DATA_BLOCK "IMAC_MOTOR2_RECORD"
TITLE =  MOTOR2_RECORD
AUTHOR : HottendU
FAMILY : IMAC
VERSION : 0.2


  STRUCT
   MOTOR2_No001 : STRUCT
    System : WORD ;
    CmdOS : WORD ;
    MirrorCmdOS : WORD ;
    Test : WORD ;
    AlarmOS : WORD ;
    StatusOS : WORD ;
    SysStatusOS : WORD ;
    Status1 : WORD ;
    Status2 : WORD ;
    Status3 : BYTE ;
    InputEdges : BYTE ;
    AutoEdges : WORD ;
    DataTimeCmd : STRUCT
     StartTime : DINT ;
     StartEdge : BOOL ;
    END_STRUCT ;
    DataTimeChg12 : STRUCT
     StartTime : DINT ;
     StartEdge : BOOL ;
    END_STRUCT ;
    DataTimeChg21 : STRUCT
     StartTime : DINT ;
     StartEdge : BOOL ;
    END_STRUCT ;
    DataTimeBlackout : STRUCT
     StartTime : DINT ;
     StartEdge : BOOL ;
    END_STRUCT ;
    DataTimeActFault : STRUCT
     StartTime : DINT ;
     StartEdge : BOOL ;
    END_STRUCT ;
    DataTimeExtFault : STRUCT
     StartTime : DINT ;
     StartEdge : BOOL ;
    END_STRUCT ;
    DataTimeFeedback : STRUCT
     StartTime : DINT ;
     StartEdge : BOOL ;
    END_STRUCT ;
    DataTimeAutoAl : STRUCT
     StartTime : DINT ;
     StartEdge : BOOL ;
    END_STRUCT ;
    PCONF : STRUCT 	//// PCONF MOTOR2 - Instance 001
     Modeswitches : STRUCT
      M0_ConstantOut : BOOL  := TRUE;	// Constant Output MST1 MST2 MSTO (1); Feedback depended Output Anst. (0)
      M1_AutoManLoc : BOOL  := TRUE;	// AUTO/ MANUAL/ LOCAL (1); MANUAL/ LOCAL (0)
      M2_NoActFeedFault : BOOL ;	// No Action- and Non-Feedback fault(1),
      M3_NoStopIfFault : BOOL  := TRUE;	// No Stop-Signal if Failure occurs (1)
      M4_RestrtAftBlack : BOOL  := TRUE;	// Restart after Blackout (1)
      M5_ResetOSonly : BOOL  := TRUE;	// Reset Alarm only with RESET from OS (1); RESET and START/STOP-Command (0)
      M6_CmdTimeDly : BOOL ;	// Command Time Delay aktiv (1)
      M7_Chg12viaStop : BOOL ;	// Change from 1->2 via STOP(1)
      M8_Chg21viaStop : BOOL ;	// Change from 2->1 via STOP(1)
      M9_StopIfAutoFail : BOOL ;	// NO AVAIL Direct Stop if Auto Failure (1)
      M10_LockBlockCmd : BOOL ;	// Lock blocksCommands
      sw11 : BOOL ;
      sw12 : BOOL ;
      sw13 : BOOL ;
      sw14 : BOOL ;
      sw15 : BOOL ;	//
     END_STRUCT ;
     DlyTCmd : TIME ;	// Setpoint Command time delay
     DlyTBlackout : TIME  := T#30S;	// Setpoint blackout time delay
     DlyTExtFault : TIME  := T#2S;	// Setpoint external fault delay
     DlyTFeedback : TIME  := T#1S;	// Setpoint feedback fault delay
     DlyTActFault : TIME  := T#5S;	// Setpoint Action Fault delay
     DlyTAutoAl : TIME  := T#3S;	// Setpoint auto alarm delay
     DlyTRestart : TIME ;	// No AVAIL Setpoint restart after blackout delay
     DlyTChg12 : TIME  := T#500MS;	// Setpoint Waiting Delay 1->2
     DlyTChg21 : TIME  := T#500MS;	// Setpoint Waiting Delay 2->1
    END_STRUCT ;
   END_STRUCT ;
   MOTOR2_No002 : STRUCT
    System : WORD ;
    CmdOS : WORD ;
    MirrorCmdOS : WORD ;
    Test : WORD ;
    AlarmOS : WORD ;
    StatusOS : WORD ;
    SysStatusOS : WORD ;
    Status1 : WORD ;
    Status2 : WORD ;
    Status3 : BYTE ;
    InputEdges : BYTE ;
    AutoEdges : WORD ;
    DataTimeCmd : STRUCT
     StartTime : DINT ;
     StartEdge : BOOL ;
    END_STRUCT ;
    DataTimeChg12 : STRUCT
     StartTime : DINT ;
     StartEdge : BOOL ;
    END_STRUCT ;
    DataTimeChg21 : STRUCT
     StartTime : DINT ;
     StartEdge : BOOL ;
    END_STRUCT ;
    DataTimeBlackout : STRUCT
     StartTime : DINT ;
     StartEdge : BOOL ;
    END_STRUCT ;
    DataTimeActFault : STRUCT
     StartTime : DINT ;
     StartEdge : BOOL ;
    END_STRUCT ;
    DataTimeExtFault : STRUCT
     StartTime : DINT ;
     StartEdge : BOOL ;
    END_STRUCT ;
    DataTimeFeedback : STRUCT
     StartTime : DINT ;
     StartEdge : BOOL ;
    END_STRUCT ;
    DataTimeAutoAl : STRUCT
     StartTime : DINT ;
     StartEdge : BOOL ;
    END_STRUCT ;
    PCONF : STRUCT 	//// PCONF MOTOR1 - Instance 002
     Modeswitches : STRUCT
      M0_ConstantOut : BOOL  := TRUE;	// Constant Output MST1 MST2 MSTO (1); Feedback depended Output Anst. (0)
      M1_AutoManLoc : BOOL  := TRUE;	// AUTO/ MANUAL/ LOCAL (1); MANUAL/ LOCAL (0)
      M2_NoActFeedFault : BOOL ;	// No Action- and Non-Feedback fault(1),
      M3_NoStopIfFault : BOOL  := TRUE;	// No Stop-Signal if Failure occurs (1)
      M4_RestrtAftBlack : BOOL  := TRUE;	// Restart after Blackout (1)
      M5_ResetOSonly : BOOL  := TRUE;	// Reset Alarm only with RESET from OS (1); RESET and START/STOP-Command (0)
      M6_CmdTimeDly : BOOL ;	// Command Time Delay aktiv (1)
      M7_Chg12viaStop : BOOL ;	// Change from 1->2 via STOP(1)
      M8_Chg21viaStop : BOOL ;	// Change from 2->1 via STOP(1)
      M9_StopIfAutoFail : BOOL ;	// NO AVAIL Direct Stop if Auto Failure (1)
      M10_LockBlockCmd : BOOL ;	// Lock blocksCommands
      sw11 : BOOL ;
      sw12 : BOOL ;
      sw13 : BOOL ;
      sw14 : BOOL ;
      sw15 : BOOL ;	//
     END_STRUCT ;
     DlyTCmd : TIME ;	// Setpoint Command time delay
     DlyTBlackout : TIME  := T#30S;	// Setpoint blackout time delay
     DlyTExtFault : TIME  := T#2S;	// Setpoint external fault delay
     DlyTFeedback : TIME  := T#1S;	// Setpoint feedback fault delay
     DlyTActFault : TIME  := T#5S;	// Setpoint Action Fault delay
     DlyTAutoAl : TIME  := T#3S;	// Setpoint auto alarm delay
     DlyTRestart : TIME ;	// No AVAIL Setpoint restart after blackout delay
     DlyTChg12 : TIME  := T#500MS;	// Setpoint Waiting Delay 1->2
     DlyTChg21 : TIME  := T#500MS;	// Setpoint Waiting Delay 2->1
    END_STRUCT ;
   END_STRUCT ;
   MOTOR2_No003 : STRUCT
    System : WORD ;
    CmdOS : WORD ;
    MirrorCmdOS : WORD ;
    Test : WORD ;
    AlarmOS : WORD ;
    StatusOS : WORD ;
    SysStatusOS : WORD ;
    Status1 : WORD ;
    Status2 : WORD ;
    Status3 : BYTE ;
    InputEdges : BYTE ;
    AutoEdges : WORD ;
    DataTimeCmd : STRUCT
     StartTime : DINT ;
     StartEdge : BOOL ;
    END_STRUCT ;
    DataTimeChg12 : STRUCT
     StartTime : DINT ;
     StartEdge : BOOL ;
    END_STRUCT ;
    DataTimeChg21 : STRUCT
     StartTime : DINT ;
     StartEdge : BOOL ;
    END_STRUCT ;
    DataTimeBlackout : STRUCT
     StartTime : DINT ;
     StartEdge : BOOL ;
    END_STRUCT ;
    DataTimeActFault : STRUCT
     StartTime : DINT ;
     StartEdge : BOOL ;
    END_STRUCT ;
    DataTimeExtFault : STRUCT
     StartTime : DINT ;
     StartEdge : BOOL ;
    END_STRUCT ;
    DataTimeFeedback : STRUCT
     StartTime : DINT ;
     StartEdge : BOOL ;
    END_STRUCT ;
    DataTimeAutoAl : STRUCT
     StartTime : DINT ;
     StartEdge : BOOL ;
    END_STRUCT ;
    PCONF : STRUCT 	//// PCONF MOTOR1 - Instance 003
     Modeswitches : STRUCT
      M0_ConstantOut : BOOL  := TRUE;	// Constant Output MST1 MST2 MSTO (1); Feedback depended Output Anst. (0)
      M1_AutoManLoc : BOOL  := TRUE;	// AUTO/ MANUAL/ LOCAL (1); MANUAL/ LOCAL (0)
      M2_NoActFeedFault : BOOL ;	// No Action- and Non-Feedback fault(1),
      M3_NoStopIfFault : BOOL  := TRUE;	// No Stop-Signal if Failure occurs (1)
      M4_RestrtAftBlack : BOOL  := TRUE;	// Restart after Blackout (1)
      M5_ResetOSonly : BOOL  := TRUE;	// Reset Alarm only with RESET from OS (1); RESET and START/STOP-Command (0)
      M6_CmdTimeDly : BOOL ;	// Command Time Delay aktiv (1)
      M7_Chg12viaStop : BOOL ;	// Change from 1->2 via STOP(1)
      M8_Chg21viaStop : BOOL ;	// Change from 2->1 via STOP(1)
      M9_StopIfAutoFail : BOOL ;	// NO AVAIL Direct Stop if Auto Failure (1)
      M10_LockBlockCmd : BOOL ;	// Lock blocksCommands
      sw11 : BOOL ;
      sw12 : BOOL ;
      sw13 : BOOL ;
      sw14 : BOOL ;
      sw15 : BOOL ;	//
     END_STRUCT ;
     DlyTCmd : TIME ;	// Setpoint Command time delay
     DlyTBlackout : TIME  := T#30S;	// Setpoint blackout time delay
     DlyTExtFault : TIME  := T#2S;	// Setpoint external fault delay
     DlyTFeedback : TIME  := T#1S;	// Setpoint feedback fault delay
     DlyTActFault : TIME  := T#5S;	// Setpoint Action Fault delay
     DlyTAutoAl : TIME  := T#3S;	// Setpoint auto alarm delay
     DlyTRestart : TIME ;	// No AVAIL Setpoint restart after blackout delay
     DlyTChg12 : TIME  := T#500MS;	// Setpoint Waiting Delay 1->2
     DlyTChg21 : TIME  := T#500MS;	// Setpoint Waiting Delay 2->1
    END_STRUCT ;
   END_STRUCT ;
   MOTOR2_No0004 : STRUCT
    System : WORD ;
    CmdOS : WORD ;
    MirrorCmdOS : WORD ;
    Test : WORD ;
    AlarmOS : WORD ;
    StatusOS : WORD ;
    SysStatusOS : WORD ;
    Status1 : WORD ;
    Status2 : WORD ;
    Status3 : BYTE ;
    InputEdges : BYTE ;
    AutoEdges : WORD ;
    DataTimeCmd : STRUCT
     StartTime : DINT ;
     StartEdge : BOOL ;
    END_STRUCT ;
    DataTimeChg12 : STRUCT
     StartTime : DINT ;
     StartEdge : BOOL ;
    END_STRUCT ;
    DataTimeChg21 : STRUCT
     StartTime : DINT ;
     StartEdge : BOOL ;
    END_STRUCT ;
    DataTimeBlackout : STRUCT
     StartTime : DINT ;
     StartEdge : BOOL ;
    END_STRUCT ;
    DataTimeActFault : STRUCT
     StartTime : DINT ;
     StartEdge : BOOL ;
    END_STRUCT ;
    DataTimeExtFault : STRUCT
     StartTime : DINT ;
     StartEdge : BOOL ;
    END_STRUCT ;
    DataTimeFeedback : STRUCT
     StartTime : DINT ;
     StartEdge : BOOL ;
    END_STRUCT ;
    DataTimeAutoAl : STRUCT
     StartTime : DINT ;
     StartEdge : BOOL ;
    END_STRUCT ;
    PCONF : STRUCT 	//// PCONF MOTOR1 - Instance 004
     Modeswitches : STRUCT
      M0_ConstantOut : BOOL ;	// Constant Output MST1 MST2 MSTO (1); Feedback depended Output Anst. (0)
      M1_AutoManLoc : BOOL ;	// AUTO/ MANUAL/ LOCAL (1); MANUAL/ LOCAL (0)
      M2_NoActFeedFault : BOOL ;	// No Action- and Non-Feedback fault(1),
      M3_NoStopIfFault : BOOL ;	// No Stop-Signal if Failure occurs (1)
      M4_RestrtAftBlack : BOOL ;	// Restart after Blackout (1)
      M5_ResetOSonly : BOOL ;	// Reset Alarm only with RESET from OS (1); RESET and START/STOP-Command (0)
      M6_CmdTimeDly : BOOL ;	// Command Time Delay aktiv (1)
      M7_Chg12viaStop : BOOL ;	// Change from 1->2 via STOP(1)
      M8_Chg21viaStop : BOOL ;	// Change from 2->1 via STOP(1)
      M9_StopIfAutoFail : BOOL ;	// NO AVAIL Direct Stop if Auto Failure (1)
      M10_LockBlockCmd : BOOL ;	// Lock blocksCommands
      sw11 : BOOL ;
      sw12 : BOOL ;
      sw13 : BOOL ;
      sw14 : BOOL ;
      sw15 : BOOL ;	//
     END_STRUCT ;
     DlyTCmd : TIME ;	// Setpoint Command time delay
     DlyTBlackout : TIME ;	// Setpoint blackout time delay
     DlyTExtFault : TIME ;	// Setpoint external fault delay
     DlyTFeedback : TIME ;	// Setpoint feedback fault delay
     DlyTActFault : TIME ;	// Setpoint Action Fault delay
     DlyTAutoAl : TIME ;	// Setpoint auto alarm delay
     DlyTRestart : TIME ;	// No AVAIL Setpoint restart after blackout delay
     DlyTChg12 : TIME ;	// Setpoint Waiting Delay 1->2
     DlyTChg21 : TIME ;	// Setpoint Waiting Delay 2->1
    END_STRUCT ;
   END_STRUCT ;
   MOTOR2_No005 : STRUCT
    System : WORD ;
    CmdOS : WORD ;
    MirrorCmdOS : WORD ;
    Test : WORD ;
    AlarmOS : WORD ;
    StatusOS : WORD ;
    SysStatusOS : WORD ;
    Status1 : WORD ;
    Status2 : WORD ;
    Status3 : BYTE ;
    InputEdges : BYTE ;
    AutoEdges : WORD ;
    DataTimeCmd : STRUCT
     StartTime : DINT ;
     StartEdge : BOOL ;
    END_STRUCT ;
    DataTimeChg12 : STRUCT
     StartTime : DINT ;
     StartEdge : BOOL ;
    END_STRUCT ;
    DataTimeChg21 : STRUCT
     StartTime : DINT ;
     StartEdge : BOOL ;
    END_STRUCT ;
    DataTimeBlackout : STRUCT
     StartTime : DINT ;
     StartEdge : BOOL ;
    END_STRUCT ;
    DataTimeActFault : STRUCT
     StartTime : DINT ;
     StartEdge : BOOL ;
    END_STRUCT ;
    DataTimeExtFault : STRUCT
     StartTime : DINT ;
     StartEdge : BOOL ;
    END_STRUCT ;
    DataTimeFeedback : STRUCT
     StartTime : DINT ;
     StartEdge : BOOL ;
    END_STRUCT ;
    DataTimeAutoAl : STRUCT
     StartTime : DINT ;
     StartEdge : BOOL ;
    END_STRUCT ;
    PCONF : STRUCT 	//// PCONF MOTOR1 - Instance 005
     Modeswitches : STRUCT
      M0_ConstantOut : BOOL ;	// Constant Output MST1 MST2 MSTO (1); Feedback depended Output Anst. (0)
      M1_AutoManLoc : BOOL ;	// AUTO/ MANUAL/ LOCAL (1); MANUAL/ LOCAL (0)
      M2_NoActFeedFault : BOOL ;	// No Action- and Non-Feedback fault(1),
      M3_NoStopIfFault : BOOL ;	// No Stop-Signal if Failure occurs (1)
      M4_RestrtAftBlack : BOOL ;	// Restart after Blackout (1)
      M5_ResetOSonly : BOOL ;	// Reset Alarm only with RESET from OS (1); RESET and START/STOP-Command (0)
      M6_CmdTimeDly : BOOL ;	// Command Time Delay aktiv (1)
      M7_Chg12viaStop : BOOL ;	// Change from 1->2 via STOP(1)
      M8_Chg21viaStop : BOOL ;	// Change from 2->1 via STOP(1)
      M9_StopIfAutoFail : BOOL ;	// NO AVAIL Direct Stop if Auto Failure (1)
      M10_LockBlockCmd : BOOL ;	// Lock blocksCommands
      sw11 : BOOL ;
      sw12 : BOOL ;
      sw13 : BOOL ;
      sw14 : BOOL ;
      sw15 : BOOL ;	//
     END_STRUCT ;
     DlyTCmd : TIME ;	// Setpoint Command time delay
     DlyTBlackout : TIME ;	// Setpoint blackout time delay
     DlyTExtFault : TIME ;	// Setpoint external fault delay
     DlyTFeedback : TIME ;	// Setpoint feedback fault delay
     DlyTActFault : TIME ;	// Setpoint Action Fault delay
     DlyTAutoAl : TIME ;	// Setpoint auto alarm delay
     DlyTRestart : TIME ;	// No AVAIL Setpoint restart after blackout delay
     DlyTChg12 : TIME ;	// Setpoint Waiting Delay 1->2
     DlyTChg21 : TIME ;	// Setpoint Waiting Delay 2->1
    END_STRUCT ;
   END_STRUCT ;
   MOTOR2_No006 : STRUCT
    System : WORD ;
    CmdOS : WORD ;
    MirrorCmdOS : WORD ;
    Test : WORD ;
    AlarmOS : WORD ;
    StatusOS : WORD ;
    SysStatusOS : WORD ;
    Status1 : WORD ;
    Status2 : WORD ;
    Status3 : BYTE ;
    InputEdges : BYTE ;
    AutoEdges : WORD ;
    DataTimeCmd : STRUCT
     StartTime : DINT ;
     StartEdge : BOOL ;
    END_STRUCT ;
    DataTimeChg12 : STRUCT
     StartTime : DINT ;
     StartEdge : BOOL ;
    END_STRUCT ;
    DataTimeChg21 : STRUCT
     StartTime : DINT ;
     StartEdge : BOOL ;
    END_STRUCT ;
    DataTimeBlackout : STRUCT
     StartTime : DINT ;
     StartEdge : BOOL ;
    END_STRUCT ;
    DataTimeActFault : STRUCT
     StartTime : DINT ;
     StartEdge : BOOL ;
    END_STRUCT ;
    DataTimeExtFault : STRUCT
     StartTime : DINT ;
     StartEdge : BOOL ;
    END_STRUCT ;
    DataTimeFeedback : STRUCT
     StartTime : DINT ;
     StartEdge : BOOL ;
    END_STRUCT ;
    DataTimeAutoAl : STRUCT
     StartTime : DINT ;
     StartEdge : BOOL ;
    END_STRUCT ;
    PCONF : STRUCT 	//// PCONF MOTOR1 - Instance 006
     Modeswitches : STRUCT
      M0_ConstantOut : BOOL ;	// Constant Output MST1 MST2 MSTO (1); Feedback depended Output Anst. (0)
      M1_AutoManLoc : BOOL ;	// AUTO/ MANUAL/ LOCAL (1); MANUAL/ LOCAL (0)
      M2_NoActFeedFault : BOOL ;	// No Action- and Non-Feedback fault(1),
      M3_NoStopIfFault : BOOL ;	// No Stop-Signal if Failure occurs (1)
      M4_RestrtAftBlack : BOOL ;	// Restart after Blackout (1)
      M5_ResetOSonly : BOOL ;	// Reset Alarm only with RESET from OS (1); RESET and START/STOP-Command (0)
      M6_CmdTimeDly : BOOL ;	// Command Time Delay aktiv (1)
      M7_Chg12viaStop : BOOL ;	// Change from 1->2 via STOP(1)
      M8_Chg21viaStop : BOOL ;	// Change from 2->1 via STOP(1)
      M9_StopIfAutoFail : BOOL ;	// NO AVAIL Direct Stop if Auto Failure (1)
      M10_LockBlockCmd : BOOL ;	// Lock blocksCommands
      sw11 : BOOL ;
      sw12 : BOOL ;
      sw13 : BOOL ;
      sw14 : BOOL ;
      sw15 : BOOL ;	//
     END_STRUCT ;
     DlyTCmd : TIME ;	// Setpoint Command time delay
     DlyTBlackout : TIME ;	// Setpoint blackout time delay
     DlyTExtFault : TIME ;	// Setpoint external fault delay
     DlyTFeedback : TIME ;	// Setpoint feedback fault delay
     DlyTActFault : TIME ;	// Setpoint Action Fault delay
     DlyTAutoAl : TIME ;	// Setpoint auto alarm delay
     DlyTRestart : TIME ;	// No AVAIL Setpoint restart after blackout delay
     DlyTChg12 : TIME ;	// Setpoint Waiting Delay 1->2
     DlyTChg21 : TIME ;	// Setpoint Waiting Delay 2->1
    END_STRUCT ;
   END_STRUCT ;
   MOTOR2_No007 : STRUCT
    System : WORD ;
    CmdOS : WORD ;
    MirrorCmdOS : WORD ;
    Test : WORD ;
    AlarmOS : WORD ;
    StatusOS : WORD ;
    SysStatusOS : WORD ;
    Status1 : WORD ;
    Status2 : WORD ;
    Status3 : BYTE ;
    InputEdges : BYTE ;
    AutoEdges : WORD ;
    DataTimeCmd : STRUCT
     StartTime : DINT ;
     StartEdge : BOOL ;
    END_STRUCT ;
    DataTimeChg12 : STRUCT
     StartTime : DINT ;
     StartEdge : BOOL ;
    END_STRUCT ;
    DataTimeChg21 : STRUCT
     StartTime : DINT ;
     StartEdge : BOOL ;
    END_STRUCT ;
    DataTimeBlackout : STRUCT
     StartTime : DINT ;
     StartEdge : BOOL ;
    END_STRUCT ;
    DataTimeActFault : STRUCT
     StartTime : DINT ;
     StartEdge : BOOL ;
    END_STRUCT ;
    DataTimeExtFault : STRUCT
     StartTime : DINT ;
     StartEdge : BOOL ;
    END_STRUCT ;
    DataTimeFeedback : STRUCT
     StartTime : DINT ;
     StartEdge : BOOL ;
    END_STRUCT ;
    DataTimeAutoAl : STRUCT
     StartTime : DINT ;
     StartEdge : BOOL ;
    END_STRUCT ;
    PCONF : STRUCT 	//// PCONF MOTOR1 - Instance 007
     Modeswitches : STRUCT
      M0_ConstantOut : BOOL ;	// Constant Output MST1 MST2 MSTO (1); Feedback depended Output Anst. (0)
      M1_AutoManLoc : BOOL ;	// AUTO/ MANUAL/ LOCAL (1); MANUAL/ LOCAL (0)
      M2_NoActFeedFault : BOOL ;	// No Action- and Non-Feedback fault(1),
      M3_NoStopIfFault : BOOL ;	// No Stop-Signal if Failure occurs (1)
      M4_RestrtAftBlack : BOOL ;	// Restart after Blackout (1)
      M5_ResetOSonly : BOOL ;	// Reset Alarm only with RESET from OS (1); RESET and START/STOP-Command (0)
      M6_CmdTimeDly : BOOL ;	// Command Time Delay aktiv (1)
      M7_Chg12viaStop : BOOL ;	// Change from 1->2 via STOP(1)
      M8_Chg21viaStop : BOOL ;	// Change from 2->1 via STOP(1)
      M9_StopIfAutoFail : BOOL ;	// NO AVAIL Direct Stop if Auto Failure (1)
      M10_LockBlockCmd : BOOL ;	// Lock blocksCommands
      sw11 : BOOL ;
      sw12 : BOOL ;
      sw13 : BOOL ;
      sw14 : BOOL ;
      sw15 : BOOL ;	//
     END_STRUCT ;
     DlyTCmd : TIME ;	// Setpoint Command time delay
     DlyTBlackout : TIME ;	// Setpoint blackout time delay
     DlyTExtFault : TIME ;	// Setpoint external fault delay
     DlyTFeedback : TIME ;	// Setpoint feedback fault delay
     DlyTActFault : TIME ;	// Setpoint Action Fault delay
     DlyTAutoAl : TIME ;	// Setpoint auto alarm delay
     DlyTRestart : TIME ;	// No AVAIL Setpoint restart after blackout delay
     DlyTChg12 : TIME ;	// Setpoint Waiting Delay 1->2
     DlyTChg21 : TIME ;	// Setpoint Waiting Delay 2->1
    END_STRUCT ;
   END_STRUCT ;
   MOTOR2_No008 : STRUCT
    System : WORD ;
    CmdOS : WORD ;
    MirrorCmdOS : WORD ;
    Test : WORD ;
    AlarmOS : WORD ;
    StatusOS : WORD ;
    SysStatusOS : WORD ;
    Status1 : WORD ;
    Status2 : WORD ;
    Status3 : BYTE ;
    InputEdges : BYTE ;
    AutoEdges : WORD ;
    DataTimeCmd : STRUCT
     StartTime : DINT ;
     StartEdge : BOOL ;
    END_STRUCT ;
    DataTimeChg12 : STRUCT
     StartTime : DINT ;
     StartEdge : BOOL ;
    END_STRUCT ;
    DataTimeChg21 : STRUCT
     StartTime : DINT ;
     StartEdge : BOOL ;
    END_STRUCT ;
    DataTimeBlackout : STRUCT
     StartTime : DINT ;
     StartEdge : BOOL ;
    END_STRUCT ;
    DataTimeActFault : STRUCT
     StartTime : DINT ;
     StartEdge : BOOL ;
    END_STRUCT ;
    DataTimeExtFault : STRUCT
     StartTime : DINT ;
     StartEdge : BOOL ;
    END_STRUCT ;
    DataTimeFeedback : STRUCT
     StartTime : DINT ;
     StartEdge : BOOL ;
    END_STRUCT ;
    DataTimeAutoAl : STRUCT
     StartTime : DINT ;
     StartEdge : BOOL ;
    END_STRUCT ;
    PCONF : STRUCT 	//// PCONF MOTOR1 - Instance 008
     Modeswitches : STRUCT
      M0_ConstantOut : BOOL ;	// Constant Output MST1 MST2 MSTO (1); Feedback depended Output Anst. (0)
      M1_AutoManLoc : BOOL ;	// AUTO/ MANUAL/ LOCAL (1); MANUAL/ LOCAL (0)
      M2_NoActFeedFault : BOOL ;	// No Action- and Non-Feedback fault(1),
      M3_NoStopIfFault : BOOL ;	// No Stop-Signal if Failure occurs (1)
      M4_RestrtAftBlack : BOOL ;	// Restart after Blackout (1)
      M5_ResetOSonly : BOOL ;	// Reset Alarm only with RESET from OS (1); RESET and START/STOP-Command (0)
      M6_CmdTimeDly : BOOL ;	// Command Time Delay aktiv (1)
      M7_Chg12viaStop : BOOL ;	// Change from 1->2 via STOP(1)
      M8_Chg21viaStop : BOOL ;	// Change from 2->1 via STOP(1)
      M9_StopIfAutoFail : BOOL ;	// NO AVAIL Direct Stop if Auto Failure (1)
      M10_LockBlockCmd : BOOL ;	// Lock blocksCommands
      sw11 : BOOL ;
      sw12 : BOOL ;
      sw13 : BOOL ;
      sw14 : BOOL ;
      sw15 : BOOL ;	//
     END_STRUCT ;
     DlyTCmd : TIME ;	// Setpoint Command time delay
     DlyTBlackout : TIME ;	// Setpoint blackout time delay
     DlyTExtFault : TIME ;	// Setpoint external fault delay
     DlyTFeedback : TIME ;	// Setpoint feedback fault delay
     DlyTActFault : TIME ;	// Setpoint Action Fault delay
     DlyTAutoAl : TIME ;	// Setpoint auto alarm delay
     DlyTRestart : TIME ;	// No AVAIL Setpoint restart after blackout delay
     DlyTChg12 : TIME ;	// Setpoint Waiting Delay 1->2
     DlyTChg21 : TIME ;	// Setpoint Waiting Delay 2->1
    END_STRUCT ;
   END_STRUCT ;
   MOTOR2_No009 : STRUCT
    System : WORD ;
    CmdOS : WORD ;
    MirrorCmdOS : WORD ;
    Test : WORD ;
    AlarmOS : WORD ;
    StatusOS : WORD ;
    SysStatusOS : WORD ;
    Status1 : WORD ;
    Status2 : WORD ;
    Status3 : BYTE ;
    InputEdges : BYTE ;
    AutoEdges : WORD ;
    DataTimeCmd : STRUCT
     StartTime : DINT ;
     StartEdge : BOOL ;
    END_STRUCT ;
    DataTimeChg12 : STRUCT
     StartTime : DINT ;
     StartEdge : BOOL ;
    END_STRUCT ;
    DataTimeChg21 : STRUCT
     StartTime : DINT ;
     StartEdge : BOOL ;
    END_STRUCT ;
    DataTimeBlackout : STRUCT
     StartTime : DINT ;
     StartEdge : BOOL ;
    END_STRUCT ;
    DataTimeActFault : STRUCT
     StartTime : DINT ;
     StartEdge : BOOL ;
    END_STRUCT ;
    DataTimeExtFault : STRUCT
     StartTime : DINT ;
     StartEdge : BOOL ;
    END_STRUCT ;
    DataTimeFeedback : STRUCT
     StartTime : DINT ;
     StartEdge : BOOL ;
    END_STRUCT ;
    DataTimeAutoAl : STRUCT
     StartTime : DINT ;
     StartEdge : BOOL ;
    END_STRUCT ;
    PCONF : STRUCT 	//// PCONF MOTOR1 - Instance 009
     Modeswitches : STRUCT
      M0_ConstantOut : BOOL ;	// Constant Output MST1 MST2 MSTO (1); Feedback depended Output Anst. (0)
      M1_AutoManLoc : BOOL ;	// AUTO/ MANUAL/ LOCAL (1); MANUAL/ LOCAL (0)
      M2_NoActFeedFault : BOOL ;	// No Action- and Non-Feedback fault(1),
      M3_NoStopIfFault : BOOL ;	// No Stop-Signal if Failure occurs (1)
      M4_RestrtAftBlack : BOOL ;	// Restart after Blackout (1)
      M5_ResetOSonly : BOOL ;	// Reset Alarm only with RESET from OS (1); RESET and START/STOP-Command (0)
      M6_CmdTimeDly : BOOL ;	// Command Time Delay aktiv (1)
      M7_Chg12viaStop : BOOL ;	// Change from 1->2 via STOP(1)
      M8_Chg21viaStop : BOOL ;	// Change from 2->1 via STOP(1)
      M9_StopIfAutoFail : BOOL ;	// NO AVAIL Direct Stop if Auto Failure (1)
      M10_LockBlockCmd : BOOL ;	// Lock blocksCommands
      sw11 : BOOL ;
      sw12 : BOOL ;
      sw13 : BOOL ;
      sw14 : BOOL ;
      sw15 : BOOL ;	//
     END_STRUCT ;
     DlyTCmd : TIME ;	// Setpoint Command time delay
     DlyTBlackout : TIME ;	// Setpoint blackout time delay
     DlyTExtFault : TIME ;	// Setpoint external fault delay
     DlyTFeedback : TIME ;	// Setpoint feedback fault delay
     DlyTActFault : TIME ;	// Setpoint Action Fault delay
     DlyTAutoAl : TIME ;	// Setpoint auto alarm delay
     DlyTRestart : TIME ;	// No AVAIL Setpoint restart after blackout delay
     DlyTChg12 : TIME ;	// Setpoint Waiting Delay 1->2
     DlyTChg21 : TIME ;	// Setpoint Waiting Delay 2->1
    END_STRUCT ;
   END_STRUCT ;
   MOTOR2_No010 : STRUCT
    System : WORD ;
    CmdOS : WORD ;
    MirrorCmdOS : WORD ;
    Test : WORD ;
    AlarmOS : WORD ;
    StatusOS : WORD ;
    SysStatusOS : WORD ;
    Status1 : WORD ;
    Status2 : WORD ;
    Status3 : BYTE ;
    InputEdges : BYTE ;
    AutoEdges : WORD ;
    DataTimeCmd : STRUCT
     StartTime : DINT ;
     StartEdge : BOOL ;
    END_STRUCT ;
    DataTimeChg12 : STRUCT
     StartTime : DINT ;
     StartEdge : BOOL ;
    END_STRUCT ;
    DataTimeChg21 : STRUCT
     StartTime : DINT ;
     StartEdge : BOOL ;
    END_STRUCT ;
    DataTimeBlackout : STRUCT
     StartTime : DINT ;
     StartEdge : BOOL ;
    END_STRUCT ;
    DataTimeActFault : STRUCT
     StartTime : DINT ;
     StartEdge : BOOL ;
    END_STRUCT ;
    DataTimeExtFault : STRUCT
     StartTime : DINT ;
     StartEdge : BOOL ;
    END_STRUCT ;
    DataTimeFeedback : STRUCT
     StartTime : DINT ;
     StartEdge : BOOL ;
    END_STRUCT ;
    DataTimeAutoAl : STRUCT
     StartTime : DINT ;
     StartEdge : BOOL ;
    END_STRUCT ;
    PCONF : STRUCT 	//// PCONF MOTOR1 - Instance 010
     Modeswitches : STRUCT
      M0_ConstantOut : BOOL ;	// Constant Output MST1 MST2 MSTO (1); Feedback depended Output Anst. (0)
      M1_AutoManLoc : BOOL ;	// AUTO/ MANUAL/ LOCAL (1); MANUAL/ LOCAL (0)
      M2_NoActFeedFault : BOOL ;	// No Action- and Non-Feedback fault(1),
      M3_NoStopIfFault : BOOL ;	// No Stop-Signal if Failure occurs (1)
      M4_RestrtAftBlack : BOOL ;	// Restart after Blackout (1)
      M5_ResetOSonly : BOOL ;	// Reset Alarm only with RESET from OS (1); RESET and START/STOP-Command (0)
      M6_CmdTimeDly : BOOL ;	// Command Time Delay aktiv (1)
      M7_Chg12viaStop : BOOL ;	// Change from 1->2 via STOP(1)
      M8_Chg21viaStop : BOOL ;	// Change from 2->1 via STOP(1)
      M9_StopIfAutoFail : BOOL ;	// NO AVAIL Direct Stop if Auto Failure (1)
      M10_LockBlockCmd : BOOL ;	// Lock blocksCommands
      sw11 : BOOL ;
      sw12 : BOOL ;
      sw13 : BOOL ;
      sw14 : BOOL ;
      sw15 : BOOL ;	//
     END_STRUCT ;
     DlyTCmd : TIME ;	// Setpoint Command time delay
     DlyTBlackout : TIME ;	// Setpoint blackout time delay
     DlyTExtFault : TIME ;	// Setpoint external fault delay
     DlyTFeedback : TIME ;	// Setpoint feedback fault delay
     DlyTActFault : TIME ;	// Setpoint Action Fault delay
     DlyTAutoAl : TIME ;	// Setpoint auto alarm delay
     DlyTRestart : TIME ;	// No AVAIL Setpoint restart after blackout delay
     DlyTChg12 : TIME ;	// Setpoint Waiting Delay 1->2
     DlyTChg21 : TIME ;	// Setpoint Waiting Delay 2->1
    END_STRUCT ;
   END_STRUCT ;
   MOTOR2_No011 : STRUCT
    System : WORD ;
    CmdOS : WORD ;
    MirrorCmdOS : WORD ;
    Test : WORD ;
    AlarmOS : WORD ;
    StatusOS : WORD ;
    SysStatusOS : WORD ;
    Status1 : WORD ;
    Status2 : WORD ;
    Status3 : BYTE ;
    InputEdges : BYTE ;
    AutoEdges : WORD ;
    DataTimeCmd : STRUCT
     StartTime : DINT ;
     StartEdge : BOOL ;
    END_STRUCT ;
    DataTimeChg12 : STRUCT
     StartTime : DINT ;
     StartEdge : BOOL ;
    END_STRUCT ;
    DataTimeChg21 : STRUCT
     StartTime : DINT ;
     StartEdge : BOOL ;
    END_STRUCT ;
    DataTimeBlackout : STRUCT
     StartTime : DINT ;
     StartEdge : BOOL ;
    END_STRUCT ;
    DataTimeActFault : STRUCT
     StartTime : DINT ;
     StartEdge : BOOL ;
    END_STRUCT ;
    DataTimeExtFault : STRUCT
     StartTime : DINT ;
     StartEdge : BOOL ;
    END_STRUCT ;
    DataTimeFeedback : STRUCT
     StartTime : DINT ;
     StartEdge : BOOL ;
    END_STRUCT ;
    DataTimeAutoAl : STRUCT
     StartTime : DINT ;
     StartEdge : BOOL ;
    END_STRUCT ;
    PCONF : STRUCT 	//// PCONF MOTOR1 - Instance 011
     Modeswitches : STRUCT
      M0_ConstantOut : BOOL ;	// Constant Output MST1 MST2 MSTO (1); Feedback depended Output Anst. (0)
      M1_AutoManLoc : BOOL ;	// AUTO/ MANUAL/ LOCAL (1); MANUAL/ LOCAL (0)
      M2_NoActFeedFault : BOOL ;	// No Action- and Non-Feedback fault(1),
      M3_NoStopIfFault : BOOL ;	// No Stop-Signal if Failure occurs (1)
      M4_RestrtAftBlack : BOOL ;	// Restart after Blackout (1)
      M5_ResetOSonly : BOOL ;	// Reset Alarm only with RESET from OS (1); RESET and START/STOP-Command (0)
      M6_CmdTimeDly : BOOL ;	// Command Time Delay aktiv (1)
      M7_Chg12viaStop : BOOL ;	// Change from 1->2 via STOP(1)
      M8_Chg21viaStop : BOOL ;	// Change from 2->1 via STOP(1)
      M9_StopIfAutoFail : BOOL ;	// NO AVAIL Direct Stop if Auto Failure (1)
      M10_LockBlockCmd : BOOL ;	// Lock blocksCommands
      sw11 : BOOL ;
      sw12 : BOOL ;
      sw13 : BOOL ;
      sw14 : BOOL ;
      sw15 : BOOL ;	//
     END_STRUCT ;
     DlyTCmd : TIME ;	// Setpoint Command time delay
     DlyTBlackout : TIME ;	// Setpoint blackout time delay
     DlyTExtFault : TIME ;	// Setpoint external fault delay
     DlyTFeedback : TIME ;	// Setpoint feedback fault delay
     DlyTActFault : TIME ;	// Setpoint Action Fault delay
     DlyTAutoAl : TIME ;	// Setpoint auto alarm delay
     DlyTRestart : TIME ;	// No AVAIL Setpoint restart after blackout delay
     DlyTChg12 : TIME ;	// Setpoint Waiting Delay 1->2
     DlyTChg21 : TIME ;	// Setpoint Waiting Delay 2->1
    END_STRUCT ;
   END_STRUCT ;
   MOTOR2_No012 : STRUCT
    System : WORD ;
    CmdOS : WORD ;
    MirrorCmdOS : WORD ;
    Test : WORD ;
    AlarmOS : WORD ;
    StatusOS : WORD ;
    SysStatusOS : WORD ;
    Status1 : WORD ;
    Status2 : WORD ;
    Status3 : BYTE ;
    InputEdges : BYTE ;
    AutoEdges : WORD ;
    DataTimeCmd : STRUCT
     StartTime : DINT ;
     StartEdge : BOOL ;
    END_STRUCT ;
    DataTimeChg12 : STRUCT
     StartTime : DINT ;
     StartEdge : BOOL ;
    END_STRUCT ;
    DataTimeChg21 : STRUCT
     StartTime : DINT ;
     StartEdge : BOOL ;
    END_STRUCT ;
    DataTimeBlackout : STRUCT
     StartTime : DINT ;
     StartEdge : BOOL ;
    END_STRUCT ;
    DataTimeActFault : STRUCT
     StartTime : DINT ;
     StartEdge : BOOL ;
    END_STRUCT ;
    DataTimeExtFault : STRUCT
     StartTime : DINT ;
     StartEdge : BOOL ;
    END_STRUCT ;
    DataTimeFeedback : STRUCT
     StartTime : DINT ;
     StartEdge : BOOL ;
    END_STRUCT ;
    DataTimeAutoAl : STRUCT
     StartTime : DINT ;
     StartEdge : BOOL ;
    END_STRUCT ;
    PCONF : STRUCT 	//// PCONF MOTOR1 - Instance 012
     Modeswitches : STRUCT
      M0_ConstantOut : BOOL ;	// Constant Output MST1 MST2 MSTO (1); Feedback depended Output Anst. (0)
      M1_AutoManLoc : BOOL ;	// AUTO/ MANUAL/ LOCAL (1); MANUAL/ LOCAL (0)
      M2_NoActFeedFault : BOOL ;	// No Action- and Non-Feedback fault(1),
      M3_NoStopIfFault : BOOL ;	// No Stop-Signal if Failure occurs (1)
      M4_RestrtAftBlack : BOOL ;	// Restart after Blackout (1)
      M5_ResetOSonly : BOOL ;	// Reset Alarm only with RESET from OS (1); RESET and START/STOP-Command (0)
      M6_CmdTimeDly : BOOL ;	// Command Time Delay aktiv (1)
      M7_Chg12viaStop : BOOL ;	// Change from 1->2 via STOP(1)
      M8_Chg21viaStop : BOOL ;	// Change from 2->1 via STOP(1)
      M9_StopIfAutoFail : BOOL ;	// NO AVAIL Direct Stop if Auto Failure (1)
      M10_LockBlockCmd : BOOL ;	// Lock blocksCommands
      sw11 : BOOL ;
      sw12 : BOOL ;
      sw13 : BOOL ;
      sw14 : BOOL ;
      sw15 : BOOL ;	//
     END_STRUCT ;
     DlyTCmd : TIME ;	// Setpoint Command time delay
     DlyTBlackout : TIME ;	// Setpoint blackout time delay
     DlyTExtFault : TIME ;	// Setpoint external fault delay
     DlyTFeedback : TIME ;	// Setpoint feedback fault delay
     DlyTActFault : TIME ;	// Setpoint Action Fault delay
     DlyTAutoAl : TIME ;	// Setpoint auto alarm delay
     DlyTRestart : TIME ;	// No AVAIL Setpoint restart after blackout delay
     DlyTChg12 : TIME ;	// Setpoint Waiting Delay 1->2
     DlyTChg21 : TIME ;	// Setpoint Waiting Delay 2->1
    END_STRUCT ;
   END_STRUCT ;
   MOTOR2_No013 : STRUCT
    System : WORD ;
    CmdOS : WORD ;
    MirrorCmdOS : WORD ;
    Test : WORD ;
    AlarmOS : WORD ;
    StatusOS : WORD ;
    SysStatusOS : WORD ;
    Status1 : WORD ;
    Status2 : WORD ;
    Status3 : BYTE ;
    InputEdges : BYTE ;
    AutoEdges : WORD ;
    DataTimeCmd : STRUCT
     StartTime : DINT ;
     StartEdge : BOOL ;
    END_STRUCT ;
    DataTimeChg12 : STRUCT
     StartTime : DINT ;
     StartEdge : BOOL ;
    END_STRUCT ;
    DataTimeChg21 : STRUCT
     StartTime : DINT ;
     StartEdge : BOOL ;
    END_STRUCT ;
    DataTimeBlackout : STRUCT
     StartTime : DINT ;
     StartEdge : BOOL ;
    END_STRUCT ;
    DataTimeActFault : STRUCT
     StartTime : DINT ;
     StartEdge : BOOL ;
    END_STRUCT ;
    DataTimeExtFault : STRUCT
     StartTime : DINT ;
     StartEdge : BOOL ;
    END_STRUCT ;
    DataTimeFeedback : STRUCT
     StartTime : DINT ;
     StartEdge : BOOL ;
    END_STRUCT ;
    DataTimeAutoAl : STRUCT
     StartTime : DINT ;
     StartEdge : BOOL ;
    END_STRUCT ;
    PCONF : STRUCT 	//// PCONF MOTOR1 - Instance 013
     Modeswitches : STRUCT
      M0_ConstantOut : BOOL ;	// Constant Output MST1 MST2 MSTO (1); Feedback depended Output Anst. (0)
      M1_AutoManLoc : BOOL ;	// AUTO/ MANUAL/ LOCAL (1); MANUAL/ LOCAL (0)
      M2_NoActFeedFault : BOOL ;	// No Action- and Non-Feedback fault(1),
      M3_NoStopIfFault : BOOL ;	// No Stop-Signal if Failure occurs (1)
      M4_RestrtAftBlack : BOOL ;	// Restart after Blackout (1)
      M5_ResetOSonly : BOOL ;	// Reset Alarm only with RESET from OS (1); RESET and START/STOP-Command (0)
      M6_CmdTimeDly : BOOL ;	// Command Time Delay aktiv (1)
      M7_Chg12viaStop : BOOL ;	// Change from 1->2 via STOP(1)
      M8_Chg21viaStop : BOOL ;	// Change from 2->1 via STOP(1)
      M9_StopIfAutoFail : BOOL ;	// NO AVAIL Direct Stop if Auto Failure (1)
      M10_LockBlockCmd : BOOL ;	// Lock blocksCommands
      sw11 : BOOL ;
      sw12 : BOOL ;
      sw13 : BOOL ;
      sw14 : BOOL ;
      sw15 : BOOL ;	//
     END_STRUCT ;
     DlyTCmd : TIME ;	// Setpoint Command time delay
     DlyTBlackout : TIME ;	// Setpoint blackout time delay
     DlyTExtFault : TIME ;	// Setpoint external fault delay
     DlyTFeedback : TIME ;	// Setpoint feedback fault delay
     DlyTActFault : TIME ;	// Setpoint Action Fault delay
     DlyTAutoAl : TIME ;	// Setpoint auto alarm delay
     DlyTRestart : TIME ;	// No AVAIL Setpoint restart after blackout delay
     DlyTChg12 : TIME ;	// Setpoint Waiting Delay 1->2
     DlyTChg21 : TIME ;	// Setpoint Waiting Delay 2->1
    END_STRUCT ;
   END_STRUCT ;
   MOTOR2_No014 : STRUCT
    System : WORD ;
    CmdOS : WORD ;
    MirrorCmdOS : WORD ;
    Test : WORD ;
    AlarmOS : WORD ;
    StatusOS : WORD ;
    SysStatusOS : WORD ;
    Status1 : WORD ;
    Status2 : WORD ;
    Status3 : BYTE ;
    InputEdges : BYTE ;
    AutoEdges : WORD ;
    DataTimeCmd : STRUCT
     StartTime : DINT ;
     StartEdge : BOOL ;
    END_STRUCT ;
    DataTimeChg12 : STRUCT
     StartTime : DINT ;
     StartEdge : BOOL ;
    END_STRUCT ;
    DataTimeChg21 : STRUCT
     StartTime : DINT ;
     StartEdge : BOOL ;
    END_STRUCT ;
    DataTimeBlackout : STRUCT
     StartTime : DINT ;
     StartEdge : BOOL ;
    END_STRUCT ;
    DataTimeActFault : STRUCT
     StartTime : DINT ;
     StartEdge : BOOL ;
    END_STRUCT ;
    DataTimeExtFault : STRUCT
     StartTime : DINT ;
     StartEdge : BOOL ;
    END_STRUCT ;
    DataTimeFeedback : STRUCT
     StartTime : DINT ;
     StartEdge : BOOL ;
    END_STRUCT ;
    DataTimeAutoAl : STRUCT
     StartTime : DINT ;
     StartEdge : BOOL ;
    END_STRUCT ;
    PCONF : STRUCT 	//// PCONF MOTOR1 - Instance 014
     Modeswitches : STRUCT
      M0_ConstantOut : BOOL ;	// Constant Output MST1 MST2 MSTO (1); Feedback depended Output Anst. (0)
      M1_AutoManLoc : BOOL ;	// AUTO/ MANUAL/ LOCAL (1); MANUAL/ LOCAL (0)
      M2_NoActFeedFault : BOOL ;	// No Action- and Non-Feedback fault(1),
      M3_NoStopIfFault : BOOL ;	// No Stop-Signal if Failure occurs (1)
      M4_RestrtAftBlack : BOOL ;	// Restart after Blackout (1)
      M5_ResetOSonly : BOOL ;	// Reset Alarm only with RESET from OS (1); RESET and START/STOP-Command (0)
      M6_CmdTimeDly : BOOL ;	// Command Time Delay aktiv (1)
      M7_Chg12viaStop : BOOL ;	// Change from 1->2 via STOP(1)
      M8_Chg21viaStop : BOOL ;	// Change from 2->1 via STOP(1)
      M9_StopIfAutoFail : BOOL ;	// NO AVAIL Direct Stop if Auto Failure (1)
      M10_LockBlockCmd : BOOL ;	// Lock blocksCommands
      sw11 : BOOL ;
      sw12 : BOOL ;
      sw13 : BOOL ;
      sw14 : BOOL ;
      sw15 : BOOL ;	//
     END_STRUCT ;
     DlyTCmd : TIME ;	// Setpoint Command time delay
     DlyTBlackout : TIME ;	// Setpoint blackout time delay
     DlyTExtFault : TIME ;	// Setpoint external fault delay
     DlyTFeedback : TIME ;	// Setpoint feedback fault delay
     DlyTActFault : TIME ;	// Setpoint Action Fault delay
     DlyTAutoAl : TIME ;	// Setpoint auto alarm delay
     DlyTRestart : TIME ;	// No AVAIL Setpoint restart after blackout delay
     DlyTChg12 : TIME ;	// Setpoint Waiting Delay 1->2
     DlyTChg21 : TIME ;	// Setpoint Waiting Delay 2->1
    END_STRUCT ;
   END_STRUCT ;
   MOTOR2_No015 : STRUCT
    System : WORD ;
    CmdOS : WORD ;
    MirrorCmdOS : WORD ;
    Test : WORD ;
    AlarmOS : WORD ;
    StatusOS : WORD ;
    SysStatusOS : WORD ;
    Status1 : WORD ;
    Status2 : WORD ;
    Status3 : BYTE ;
    InputEdges : BYTE ;
    AutoEdges : WORD ;
    DataTimeCmd : STRUCT
     StartTime : DINT ;
     StartEdge : BOOL ;
    END_STRUCT ;
    DataTimeChg12 : STRUCT
     StartTime : DINT ;
     StartEdge : BOOL ;
    END_STRUCT ;
    DataTimeChg21 : STRUCT
     StartTime : DINT ;
     StartEdge : BOOL ;
    END_STRUCT ;
    DataTimeBlackout : STRUCT
     StartTime : DINT ;
     StartEdge : BOOL ;
    END_STRUCT ;
    DataTimeActFault : STRUCT
     StartTime : DINT ;
     StartEdge : BOOL ;
    END_STRUCT ;
    DataTimeExtFault : STRUCT
     StartTime : DINT ;
     StartEdge : BOOL ;
    END_STRUCT ;
    DataTimeFeedback : STRUCT
     StartTime : DINT ;
     StartEdge : BOOL ;
    END_STRUCT ;
    DataTimeAutoAl : STRUCT
     StartTime : DINT ;
     StartEdge : BOOL ;
    END_STRUCT ;
    PCONF : STRUCT 	//// PCONF MOTOR1 - Instance 015
     Modeswitches : STRUCT
      M0_ConstantOut : BOOL ;	// Constant Output MST1 MST2 MSTO (1); Feedback depended Output Anst. (0)
      M1_AutoManLoc : BOOL ;	// AUTO/ MANUAL/ LOCAL (1); MANUAL/ LOCAL (0)
      M2_NoActFeedFault : BOOL ;	// No Action- and Non-Feedback fault(1),
      M3_NoStopIfFault : BOOL ;	// No Stop-Signal if Failure occurs (1)
      M4_RestrtAftBlack : BOOL ;	// Restart after Blackout (1)
      M5_ResetOSonly : BOOL ;	// Reset Alarm only with RESET from OS (1); RESET and START/STOP-Command (0)
      M6_CmdTimeDly : BOOL ;	// Command Time Delay aktiv (1)
      M7_Chg12viaStop : BOOL ;	// Change from 1->2 via STOP(1)
      M8_Chg21viaStop : BOOL ;	// Change from 2->1 via STOP(1)
      M9_StopIfAutoFail : BOOL ;	// NO AVAIL Direct Stop if Auto Failure (1)
      M10_LockBlockCmd : BOOL ;	// Lock blocksCommands
      sw11 : BOOL ;
      sw12 : BOOL ;
      sw13 : BOOL ;
      sw14 : BOOL ;
      sw15 : BOOL ;	//
     END_STRUCT ;
     DlyTCmd : TIME ;	// Setpoint Command time delay
     DlyTBlackout : TIME ;	// Setpoint blackout time delay
     DlyTExtFault : TIME ;	// Setpoint external fault delay
     DlyTFeedback : TIME ;	// Setpoint feedback fault delay
     DlyTActFault : TIME ;	// Setpoint Action Fault delay
     DlyTAutoAl : TIME ;	// Setpoint auto alarm delay
     DlyTRestart : TIME ;	// No AVAIL Setpoint restart after blackout delay
     DlyTChg12 : TIME ;	// Setpoint Waiting Delay 1->2
     DlyTChg21 : TIME ;	// Setpoint Waiting Delay 2->1
    END_STRUCT ;
   END_STRUCT ;
   MOTOR2_No016 : STRUCT
    System : WORD ;
    CmdOS : WORD ;
    MirrorCmdOS : WORD ;
    Test : WORD ;
    AlarmOS : WORD ;
    StatusOS : WORD ;
    SysStatusOS : WORD ;
    Status1 : WORD ;
    Status2 : WORD ;
    Status3 : BYTE ;
    InputEdges : BYTE ;
    AutoEdges : WORD ;
    DataTimeCmd : STRUCT
     StartTime : DINT ;
     StartEdge : BOOL ;
    END_STRUCT ;
    DataTimeChg12 : STRUCT
     StartTime : DINT ;
     StartEdge : BOOL ;
    END_STRUCT ;
    DataTimeChg21 : STRUCT
     StartTime : DINT ;
     StartEdge : BOOL ;
    END_STRUCT ;
    DataTimeBlackout : STRUCT
     StartTime : DINT ;
     StartEdge : BOOL ;
    END_STRUCT ;
    DataTimeActFault : STRUCT
     StartTime : DINT ;
     StartEdge : BOOL ;
    END_STRUCT ;
    DataTimeExtFault : STRUCT
     StartTime : DINT ;
     StartEdge : BOOL ;
    END_STRUCT ;
    DataTimeFeedback : STRUCT
     StartTime : DINT ;
     StartEdge : BOOL ;
    END_STRUCT ;
    DataTimeAutoAl : STRUCT
     StartTime : DINT ;
     StartEdge : BOOL ;
    END_STRUCT ;
    PCONF : STRUCT 	//// PCONF MOTOR1 - Instance 016
     Modeswitches : STRUCT
      M0_ConstantOut : BOOL ;	// Constant Output MST1 MST2 MSTO (1); Feedback depended Output Anst. (0)
      M1_AutoManLoc : BOOL ;	// AUTO/ MANUAL/ LOCAL (1); MANUAL/ LOCAL (0)
      M2_NoActFeedFault : BOOL ;	// No Action- and Non-Feedback fault(1),
      M3_NoStopIfFault : BOOL ;	// No Stop-Signal if Failure occurs (1)
      M4_RestrtAftBlack : BOOL ;	// Restart after Blackout (1)
      M5_ResetOSonly : BOOL ;	// Reset Alarm only with RESET from OS (1); RESET and START/STOP-Command (0)
      M6_CmdTimeDly : BOOL ;	// Command Time Delay aktiv (1)
      M7_Chg12viaStop : BOOL ;	// Change from 1->2 via STOP(1)
      M8_Chg21viaStop : BOOL ;	// Change from 2->1 via STOP(1)
      M9_StopIfAutoFail : BOOL ;	// NO AVAIL Direct Stop if Auto Failure (1)
      M10_LockBlockCmd : BOOL ;	// Lock blocksCommands
      sw11 : BOOL ;
      sw12 : BOOL ;
      sw13 : BOOL ;
      sw14 : BOOL ;
      sw15 : BOOL ;	//
     END_STRUCT ;
     DlyTCmd : TIME ;	// Setpoint Command time delay
     DlyTBlackout : TIME ;	// Setpoint blackout time delay
     DlyTExtFault : TIME ;	// Setpoint external fault delay
     DlyTFeedback : TIME ;	// Setpoint feedback fault delay
     DlyTActFault : TIME ;	// Setpoint Action Fault delay
     DlyTAutoAl : TIME ;	// Setpoint auto alarm delay
     DlyTRestart : TIME ;	// No AVAIL Setpoint restart after blackout delay
     DlyTChg12 : TIME ;	// Setpoint Waiting Delay 1->2
     DlyTChg21 : TIME ;	// Setpoint Waiting Delay 2->1
    END_STRUCT ;
   END_STRUCT ;
   MOTOR2_No017 : STRUCT
    System : WORD ;
    CmdOS : WORD ;
    MirrorCmdOS : WORD ;
    Test : WORD ;
    AlarmOS : WORD ;
    StatusOS : WORD ;
    SysStatusOS : WORD ;
    Status1 : WORD ;
    Status2 : WORD ;
    Status3 : BYTE ;
    InputEdges : BYTE ;
    AutoEdges : WORD ;
    DataTimeCmd : STRUCT
     StartTime : DINT ;
     StartEdge : BOOL ;
    END_STRUCT ;
    DataTimeChg12 : STRUCT
     StartTime : DINT ;
     StartEdge : BOOL ;
    END_STRUCT ;
    DataTimeChg21 : STRUCT
     StartTime : DINT ;
     StartEdge : BOOL ;
    END_STRUCT ;
    DataTimeBlackout : STRUCT
     StartTime : DINT ;
     StartEdge : BOOL ;
    END_STRUCT ;
    DataTimeActFault : STRUCT
     StartTime : DINT ;
     StartEdge : BOOL ;
    END_STRUCT ;
    DataTimeExtFault : STRUCT
     StartTime : DINT ;
     StartEdge : BOOL ;
    END_STRUCT ;
    DataTimeFeedback : STRUCT
     StartTime : DINT ;
     StartEdge : BOOL ;
    END_STRUCT ;
    DataTimeAutoAl : STRUCT
     StartTime : DINT ;
     StartEdge : BOOL ;
    END_STRUCT ;
    PCONF : STRUCT 	//// PCONF MOTOR1 - Instance 017
     Modeswitches : STRUCT
      M0_ConstantOut : BOOL ;	// Constant Output MST1 MST2 MSTO (1); Feedback depended Output Anst. (0)
      M1_AutoManLoc : BOOL ;	// AUTO/ MANUAL/ LOCAL (1); MANUAL/ LOCAL (0)
      M2_NoActFeedFault : BOOL ;	// No Action- and Non-Feedback fault(1),
      M3_NoStopIfFault : BOOL ;	// No Stop-Signal if Failure occurs (1)
      M4_RestrtAftBlack : BOOL ;	// Restart after Blackout (1)
      M5_ResetOSonly : BOOL ;	// Reset Alarm only with RESET from OS (1); RESET and START/STOP-Command (0)
      M6_CmdTimeDly : BOOL ;	// Command Time Delay aktiv (1)
      M7_Chg12viaStop : BOOL ;	// Change from 1->2 via STOP(1)
      M8_Chg21viaStop : BOOL ;	// Change from 2->1 via STOP(1)
      M9_StopIfAutoFail : BOOL ;	// NO AVAIL Direct Stop if Auto Failure (1)
      M10_LockBlockCmd : BOOL ;	// Lock blocksCommands
      sw11 : BOOL ;
      sw12 : BOOL ;
      sw13 : BOOL ;
      sw14 : BOOL ;
      sw15 : BOOL ;	//
     END_STRUCT ;
     DlyTCmd : TIME ;	// Setpoint Command time delay
     DlyTBlackout : TIME ;	// Setpoint blackout time delay
     DlyTExtFault : TIME ;	// Setpoint external fault delay
     DlyTFeedback : TIME ;	// Setpoint feedback fault delay
     DlyTActFault : TIME ;	// Setpoint Action Fault delay
     DlyTAutoAl : TIME ;	// Setpoint auto alarm delay
     DlyTRestart : TIME ;	// No AVAIL Setpoint restart after blackout delay
     DlyTChg12 : TIME ;	// Setpoint Waiting Delay 1->2
     DlyTChg21 : TIME ;	// Setpoint Waiting Delay 2->1
    END_STRUCT ;
   END_STRUCT ;
   MOTOR2_No018 : STRUCT
    System : WORD ;
    CmdOS : WORD ;
    MirrorCmdOS : WORD ;
    Test : WORD ;
    AlarmOS : WORD ;
    StatusOS : WORD ;
    SysStatusOS : WORD ;
    Status1 : WORD ;
    Status2 : WORD ;
    Status3 : BYTE ;
    InputEdges : BYTE ;
    AutoEdges : WORD ;
    DataTimeCmd : STRUCT
     StartTime : DINT ;
     StartEdge : BOOL ;
    END_STRUCT ;
    DataTimeChg12 : STRUCT
     StartTime : DINT ;
     StartEdge : BOOL ;
    END_STRUCT ;
    DataTimeChg21 : STRUCT
     StartTime : DINT ;
     StartEdge : BOOL ;
    END_STRUCT ;
    DataTimeBlackout : STRUCT
     StartTime : DINT ;
     StartEdge : BOOL ;
    END_STRUCT ;
    DataTimeActFault : STRUCT
     StartTime : DINT ;
     StartEdge : BOOL ;
    END_STRUCT ;
    DataTimeExtFault : STRUCT
     StartTime : DINT ;
     StartEdge : BOOL ;
    END_STRUCT ;
    DataTimeFeedback : STRUCT
     StartTime : DINT ;
     StartEdge : BOOL ;
    END_STRUCT ;
    DataTimeAutoAl : STRUCT
     StartTime : DINT ;
     StartEdge : BOOL ;
    END_STRUCT ;
    PCONF : STRUCT 	//// PCONF MOTOR1 - Instance 018
     Modeswitches : STRUCT
      M0_ConstantOut : BOOL ;	// Constant Output MST1 MST2 MSTO (1); Feedback depended Output Anst. (0)
      M1_AutoManLoc : BOOL ;	// AUTO/ MANUAL/ LOCAL (1); MANUAL/ LOCAL (0)
      M2_NoActFeedFault : BOOL ;	// No Action- and Non-Feedback fault(1),
      M3_NoStopIfFault : BOOL ;	// No Stop-Signal if Failure occurs (1)
      M4_RestrtAftBlack : BOOL ;	// Restart after Blackout (1)
      M5_ResetOSonly : BOOL ;	// Reset Alarm only with RESET from OS (1); RESET and START/STOP-Command (0)
      M6_CmdTimeDly : BOOL ;	// Command Time Delay aktiv (1)
      M7_Chg12viaStop : BOOL ;	// Change from 1->2 via STOP(1)
      M8_Chg21viaStop : BOOL ;	// Change from 2->1 via STOP(1)
      M9_StopIfAutoFail : BOOL ;	// NO AVAIL Direct Stop if Auto Failure (1)
      M10_LockBlockCmd : BOOL ;	// Lock blocksCommands
      sw11 : BOOL ;
      sw12 : BOOL ;
      sw13 : BOOL ;
      sw14 : BOOL ;
      sw15 : BOOL ;	//
     END_STRUCT ;
     DlyTCmd : TIME ;	// Setpoint Command time delay
     DlyTBlackout : TIME ;	// Setpoint blackout time delay
     DlyTExtFault : TIME ;	// Setpoint external fault delay
     DlyTFeedback : TIME ;	// Setpoint feedback fault delay
     DlyTActFault : TIME ;	// Setpoint Action Fault delay
     DlyTAutoAl : TIME ;	// Setpoint auto alarm delay
     DlyTRestart : TIME ;	// No AVAIL Setpoint restart after blackout delay
     DlyTChg12 : TIME ;	// Setpoint Waiting Delay 1->2
     DlyTChg21 : TIME ;	// Setpoint Waiting Delay 2->1
    END_STRUCT ;
   END_STRUCT ;
   MOTOR2_No019 : STRUCT
    System : WORD ;
    CmdOS : WORD ;
    MirrorCmdOS : WORD ;
    Test : WORD ;
    AlarmOS : WORD ;
    StatusOS : WORD ;
    SysStatusOS : WORD ;
    Status1 : WORD ;
    Status2 : WORD ;
    Status3 : BYTE ;
    InputEdges : BYTE ;
    AutoEdges : WORD ;
    DataTimeCmd : STRUCT
     StartTime : DINT ;
     StartEdge : BOOL ;
    END_STRUCT ;
    DataTimeChg12 : STRUCT
     StartTime : DINT ;
     StartEdge : BOOL ;
    END_STRUCT ;
    DataTimeChg21 : STRUCT
     StartTime : DINT ;
     StartEdge : BOOL ;
    END_STRUCT ;
    DataTimeBlackout : STRUCT
     StartTime : DINT ;
     StartEdge : BOOL ;
    END_STRUCT ;
    DataTimeActFault : STRUCT
     StartTime : DINT ;
     StartEdge : BOOL ;
    END_STRUCT ;
    DataTimeExtFault : STRUCT
     StartTime : DINT ;
     StartEdge : BOOL ;
    END_STRUCT ;
    DataTimeFeedback : STRUCT
     StartTime : DINT ;
     StartEdge : BOOL ;
    END_STRUCT ;
    DataTimeAutoAl : STRUCT
     StartTime : DINT ;
     StartEdge : BOOL ;
    END_STRUCT ;
    PCONF : STRUCT 	//// PCONF MOTOR1 - Instance 019
     Modeswitches : STRUCT
      M0_ConstantOut : BOOL ;	// Constant Output MST1 MST2 MSTO (1); Feedback depended Output Anst. (0)
      M1_AutoManLoc : BOOL ;	// AUTO/ MANUAL/ LOCAL (1); MANUAL/ LOCAL (0)
      M2_NoActFeedFault : BOOL ;	// No Action- and Non-Feedback fault(1),
      M3_NoStopIfFault : BOOL ;	// No Stop-Signal if Failure occurs (1)
      M4_RestrtAftBlack : BOOL ;	// Restart after Blackout (1)
      M5_ResetOSonly : BOOL ;	// Reset Alarm only with RESET from OS (1); RESET and START/STOP-Command (0)
      M6_CmdTimeDly : BOOL ;	// Command Time Delay aktiv (1)
      M7_Chg12viaStop : BOOL ;	// Change from 1->2 via STOP(1)
      M8_Chg21viaStop : BOOL ;	// Change from 2->1 via STOP(1)
      M9_StopIfAutoFail : BOOL ;	// NO AVAIL Direct Stop if Auto Failure (1)
      M10_LockBlockCmd : BOOL ;	// Lock blocksCommands
      sw11 : BOOL ;
      sw12 : BOOL ;
      sw13 : BOOL ;
      sw14 : BOOL ;
      sw15 : BOOL ;	//
     END_STRUCT ;
     DlyTCmd : TIME ;	// Setpoint Command time delay
     DlyTBlackout : TIME ;	// Setpoint blackout time delay
     DlyTExtFault : TIME ;	// Setpoint external fault delay
     DlyTFeedback : TIME ;	// Setpoint feedback fault delay
     DlyTActFault : TIME ;	// Setpoint Action Fault delay
     DlyTAutoAl : TIME ;	// Setpoint auto alarm delay
     DlyTRestart : TIME ;	// No AVAIL Setpoint restart after blackout delay
     DlyTChg12 : TIME ;	// Setpoint Waiting Delay 1->2
     DlyTChg21 : TIME ;	// Setpoint Waiting Delay 2->1
    END_STRUCT ;
   END_STRUCT ;
   MOTOR2_No020 : STRUCT
    System : WORD ;
    CmdOS : WORD ;
    MirrorCmdOS : WORD ;
    Test : WORD ;
    AlarmOS : WORD ;
    StatusOS : WORD ;
    SysStatusOS : WORD ;
    Status1 : WORD ;
    Status2 : WORD ;
    Status3 : BYTE ;
    InputEdges : BYTE ;
    AutoEdges : WORD ;
    DataTimeCmd : STRUCT
     StartTime : DINT ;
     StartEdge : BOOL ;
    END_STRUCT ;
    DataTimeChg12 : STRUCT
     StartTime : DINT ;
     StartEdge : BOOL ;
    END_STRUCT ;
    DataTimeChg21 : STRUCT
     StartTime : DINT ;
     StartEdge : BOOL ;
    END_STRUCT ;
    DataTimeBlackout : STRUCT
     StartTime : DINT ;
     StartEdge : BOOL ;
    END_STRUCT ;
    DataTimeActFault : STRUCT
     StartTime : DINT ;
     StartEdge : BOOL ;
    END_STRUCT ;
    DataTimeExtFault : STRUCT
     StartTime : DINT ;
     StartEdge : BOOL ;
    END_STRUCT ;
    DataTimeFeedback : STRUCT
     StartTime : DINT ;
     StartEdge : BOOL ;
    END_STRUCT ;
    DataTimeAutoAl : STRUCT
     StartTime : DINT ;
     StartEdge : BOOL ;
    END_STRUCT ;
    PCONF : STRUCT 	//// PCONF MOTOR1 - Instance 020
     Modeswitches : STRUCT
      M0_ConstantOut : BOOL ;	// Constant Output MST1 MST2 MSTO (1); Feedback depended Output Anst. (0)
      M1_AutoManLoc : BOOL ;	// AUTO/ MANUAL/ LOCAL (1); MANUAL/ LOCAL (0)
      M2_NoActFeedFault : BOOL ;	// No Action- and Non-Feedback fault(1),
      M3_NoStopIfFault : BOOL ;	// No Stop-Signal if Failure occurs (1)
      M4_RestrtAftBlack : BOOL ;	// Restart after Blackout (1)
      M5_ResetOSonly : BOOL ;	// Reset Alarm only with RESET from OS (1); RESET and START/STOP-Command (0)
      M6_CmdTimeDly : BOOL ;	// Command Time Delay aktiv (1)
      M7_Chg12viaStop : BOOL ;	// Change from 1->2 via STOP(1)
      M8_Chg21viaStop : BOOL ;	// Change from 2->1 via STOP(1)
      M9_StopIfAutoFail : BOOL ;	// NO AVAIL Direct Stop if Auto Failure (1)
      M10_LockBlockCmd : BOOL ;	// Lock blocksCommands
      sw11 : BOOL ;
      sw12 : BOOL ;
      sw13 : BOOL ;
      sw14 : BOOL ;
      sw15 : BOOL ;	//
     END_STRUCT ;
     DlyTCmd : TIME ;	// Setpoint Command time delay
     DlyTBlackout : TIME ;	// Setpoint blackout time delay
     DlyTExtFault : TIME ;	// Setpoint external fault delay
     DlyTFeedback : TIME ;	// Setpoint feedback fault delay
     DlyTActFault : TIME ;	// Setpoint Action Fault delay
     DlyTAutoAl : TIME ;	// Setpoint auto alarm delay
     DlyTRestart : TIME ;	// No AVAIL Setpoint restart after blackout delay
     DlyTChg12 : TIME ;	// Setpoint Waiting Delay 1->2
     DlyTChg21 : TIME ;	// Setpoint Waiting Delay 2->1
    END_STRUCT ;
   END_STRUCT ;
   MOTOR2_No021 : STRUCT
    System : WORD ;
    CmdOS : WORD ;
    MirrorCmdOS : WORD ;
    Test : WORD ;
    AlarmOS : WORD ;
    StatusOS : WORD ;
    SysStatusOS : WORD ;
    Status1 : WORD ;
    Status2 : WORD ;
    Status3 : BYTE ;
    InputEdges : BYTE ;
    AutoEdges : WORD ;
    DataTimeCmd : STRUCT
     StartTime : DINT ;
     StartEdge : BOOL ;
    END_STRUCT ;
    DataTimeChg12 : STRUCT
     StartTime : DINT ;
     StartEdge : BOOL ;
    END_STRUCT ;
    DataTimeChg21 : STRUCT
     StartTime : DINT ;
     StartEdge : BOOL ;
    END_STRUCT ;
    DataTimeBlackout : STRUCT
     StartTime : DINT ;
     StartEdge : BOOL ;
    END_STRUCT ;
    DataTimeActFault : STRUCT
     StartTime : DINT ;
     StartEdge : BOOL ;
    END_STRUCT ;
    DataTimeExtFault : STRUCT
     StartTime : DINT ;
     StartEdge : BOOL ;
    END_STRUCT ;
    DataTimeFeedback : STRUCT
     StartTime : DINT ;
     StartEdge : BOOL ;
    END_STRUCT ;
    DataTimeAutoAl : STRUCT
     StartTime : DINT ;
     StartEdge : BOOL ;
    END_STRUCT ;
    PCONF : STRUCT 	//// PCONF MOTOR1 - Instance 021
     Modeswitches : STRUCT
      M0_ConstantOut : BOOL ;	// Constant Output MST1 MST2 MSTO (1); Feedback depended Output Anst. (0)
      M1_AutoManLoc : BOOL ;	// AUTO/ MANUAL/ LOCAL (1); MANUAL/ LOCAL (0)
      M2_NoActFeedFault : BOOL ;	// No Action- and Non-Feedback fault(1),
      M3_NoStopIfFault : BOOL ;	// No Stop-Signal if Failure occurs (1)
      M4_RestrtAftBlack : BOOL ;	// Restart after Blackout (1)
      M5_ResetOSonly : BOOL ;	// Reset Alarm only with RESET from OS (1); RESET and START/STOP-Command (0)
      M6_CmdTimeDly : BOOL ;	// Command Time Delay aktiv (1)
      M7_Chg12viaStop : BOOL ;	// Change from 1->2 via STOP(1)
      M8_Chg21viaStop : BOOL ;	// Change from 2->1 via STOP(1)
      M9_StopIfAutoFail : BOOL ;	// NO AVAIL Direct Stop if Auto Failure (1)
      M10_LockBlockCmd : BOOL ;	// Lock blocksCommands
      sw11 : BOOL ;
      sw12 : BOOL ;
      sw13 : BOOL ;
      sw14 : BOOL ;
      sw15 : BOOL ;	//
     END_STRUCT ;
     DlyTCmd : TIME ;	// Setpoint Command time delay
     DlyTBlackout : TIME ;	// Setpoint blackout time delay
     DlyTExtFault : TIME ;	// Setpoint external fault delay
     DlyTFeedback : TIME ;	// Setpoint feedback fault delay
     DlyTActFault : TIME ;	// Setpoint Action Fault delay
     DlyTAutoAl : TIME ;	// Setpoint auto alarm delay
     DlyTRestart : TIME ;	// No AVAIL Setpoint restart after blackout delay
     DlyTChg12 : TIME ;	// Setpoint Waiting Delay 1->2
     DlyTChg21 : TIME ;	// Setpoint Waiting Delay 2->1
    END_STRUCT ;
   END_STRUCT ;
   MOTOR2_No022 : STRUCT
    System : WORD ;
    CmdOS : WORD ;
    MirrorCmdOS : WORD ;
    Test : WORD ;
    AlarmOS : WORD ;
    StatusOS : WORD ;
    SysStatusOS : WORD ;
    Status1 : WORD ;
    Status2 : WORD ;
    Status3 : BYTE ;
    InputEdges : BYTE ;
    AutoEdges : WORD ;
    DataTimeCmd : STRUCT
     StartTime : DINT ;
     StartEdge : BOOL ;
    END_STRUCT ;
    DataTimeChg12 : STRUCT
     StartTime : DINT ;
     StartEdge : BOOL ;
    END_STRUCT ;
    DataTimeChg21 : STRUCT
     StartTime : DINT ;
     StartEdge : BOOL ;
    END_STRUCT ;
    DataTimeBlackout : STRUCT
     StartTime : DINT ;
     StartEdge : BOOL ;
    END_STRUCT ;
    DataTimeActFault : STRUCT
     StartTime : DINT ;
     StartEdge : BOOL ;
    END_STRUCT ;
    DataTimeExtFault : STRUCT
     StartTime : DINT ;
     StartEdge : BOOL ;
    END_STRUCT ;
    DataTimeFeedback : STRUCT
     StartTime : DINT ;
     StartEdge : BOOL ;
    END_STRUCT ;
    DataTimeAutoAl : STRUCT
     StartTime : DINT ;
     StartEdge : BOOL ;
    END_STRUCT ;
    PCONF : STRUCT 	//// PCONF MOTOR1 - Instance 022
     Modeswitches : STRUCT
      M0_ConstantOut : BOOL ;	// Constant Output MST1 MST2 MSTO (1); Feedback depended Output Anst. (0)
      M1_AutoManLoc : BOOL ;	// AUTO/ MANUAL/ LOCAL (1); MANUAL/ LOCAL (0)
      M2_NoActFeedFault : BOOL ;	// No Action- and Non-Feedback fault(1),
      M3_NoStopIfFault : BOOL ;	// No Stop-Signal if Failure occurs (1)
      M4_RestrtAftBlack : BOOL ;	// Restart after Blackout (1)
      M5_ResetOSonly : BOOL ;	// Reset Alarm only with RESET from OS (1); RESET and START/STOP-Command (0)
      M6_CmdTimeDly : BOOL ;	// Command Time Delay aktiv (1)
      M7_Chg12viaStop : BOOL ;	// Change from 1->2 via STOP(1)
      M8_Chg21viaStop : BOOL ;	// Change from 2->1 via STOP(1)
      M9_StopIfAutoFail : BOOL ;	// NO AVAIL Direct Stop if Auto Failure (1)
      M10_LockBlockCmd : BOOL ;	// Lock blocksCommands
      sw11 : BOOL ;
      sw12 : BOOL ;
      sw13 : BOOL ;
      sw14 : BOOL ;
      sw15 : BOOL ;	//
     END_STRUCT ;
     DlyTCmd : TIME ;	// Setpoint Command time delay
     DlyTBlackout : TIME ;	// Setpoint blackout time delay
     DlyTExtFault : TIME ;	// Setpoint external fault delay
     DlyTFeedback : TIME ;	// Setpoint feedback fault delay
     DlyTActFault : TIME ;	// Setpoint Action Fault delay
     DlyTAutoAl : TIME ;	// Setpoint auto alarm delay
     DlyTRestart : TIME ;	// No AVAIL Setpoint restart after blackout delay
     DlyTChg12 : TIME ;	// Setpoint Waiting Delay 1->2
     DlyTChg21 : TIME ;	// Setpoint Waiting Delay 2->1
    END_STRUCT ;
   END_STRUCT ;
   MOTOR2_No023 : STRUCT
    System : WORD ;
    CmdOS : WORD ;
    MirrorCmdOS : WORD ;
    Test : WORD ;
    AlarmOS : WORD ;
    StatusOS : WORD ;
    SysStatusOS : WORD ;
    Status1 : WORD ;
    Status2 : WORD ;
    Status3 : BYTE ;
    InputEdges : BYTE ;
    AutoEdges : WORD ;
    DataTimeCmd : STRUCT
     StartTime : DINT ;
     StartEdge : BOOL ;
    END_STRUCT ;
    DataTimeChg12 : STRUCT
     StartTime : DINT ;
     StartEdge : BOOL ;
    END_STRUCT ;
    DataTimeChg21 : STRUCT
     StartTime : DINT ;
     StartEdge : BOOL ;
    END_STRUCT ;
    DataTimeBlackout : STRUCT
     StartTime : DINT ;
     StartEdge : BOOL ;
    END_STRUCT ;
    DataTimeActFault : STRUCT
     StartTime : DINT ;
     StartEdge : BOOL ;
    END_STRUCT ;
    DataTimeExtFault : STRUCT
     StartTime : DINT ;
     StartEdge : BOOL ;
    END_STRUCT ;
    DataTimeFeedback : STRUCT
     StartTime : DINT ;
     StartEdge : BOOL ;
    END_STRUCT ;
    DataTimeAutoAl : STRUCT
     StartTime : DINT ;
     StartEdge : BOOL ;
    END_STRUCT ;
    PCONF : STRUCT 	//// PCONF MOTOR1 - Instance 023
     Modeswitches : STRUCT
      M0_ConstantOut : BOOL ;	// Constant Output MST1 MST2 MSTO (1); Feedback depended Output Anst. (0)
      M1_AutoManLoc : BOOL ;	// AUTO/ MANUAL/ LOCAL (1); MANUAL/ LOCAL (0)
      M2_NoActFeedFault : BOOL ;	// No Action- and Non-Feedback fault(1),
      M3_NoStopIfFault : BOOL ;	// No Stop-Signal if Failure occurs (1)
      M4_RestrtAftBlack : BOOL ;	// Restart after Blackout (1)
      M5_ResetOSonly : BOOL ;	// Reset Alarm only with RESET from OS (1); RESET and START/STOP-Command (0)
      M6_CmdTimeDly : BOOL ;	// Command Time Delay aktiv (1)
      M7_Chg12viaStop : BOOL ;	// Change from 1->2 via STOP(1)
      M8_Chg21viaStop : BOOL ;	// Change from 2->1 via STOP(1)
      M9_StopIfAutoFail : BOOL ;	// NO AVAIL Direct Stop if Auto Failure (1)
      M10_LockBlockCmd : BOOL ;	// Lock blocksCommands
      sw11 : BOOL ;
      sw12 : BOOL ;
      sw13 : BOOL ;
      sw14 : BOOL ;
      sw15 : BOOL ;	//
     END_STRUCT ;
     DlyTCmd : TIME ;	// Setpoint Command time delay
     DlyTBlackout : TIME ;	// Setpoint blackout time delay
     DlyTExtFault : TIME ;	// Setpoint external fault delay
     DlyTFeedback : TIME ;	// Setpoint feedback fault delay
     DlyTActFault : TIME ;	// Setpoint Action Fault delay
     DlyTAutoAl : TIME ;	// Setpoint auto alarm delay
     DlyTRestart : TIME ;	// No AVAIL Setpoint restart after blackout delay
     DlyTChg12 : TIME ;	// Setpoint Waiting Delay 1->2
     DlyTChg21 : TIME ;	// Setpoint Waiting Delay 2->1
    END_STRUCT ;
   END_STRUCT ;
   MOTOR2_No024 : STRUCT
    System : WORD ;
    CmdOS : WORD ;
    MirrorCmdOS : WORD ;
    Test : WORD ;
    AlarmOS : WORD ;
    StatusOS : WORD ;
    SysStatusOS : WORD ;
    Status1 : WORD ;
    Status2 : WORD ;
    Status3 : BYTE ;
    InputEdges : BYTE ;
    AutoEdges : WORD ;
    DataTimeCmd : STRUCT
     StartTime : DINT ;
     StartEdge : BOOL ;
    END_STRUCT ;
    DataTimeChg12 : STRUCT
     StartTime : DINT ;
     StartEdge : BOOL ;
    END_STRUCT ;
    DataTimeChg21 : STRUCT
     StartTime : DINT ;
     StartEdge : BOOL ;
    END_STRUCT ;
    DataTimeBlackout : STRUCT
     StartTime : DINT ;
     StartEdge : BOOL ;
    END_STRUCT ;
    DataTimeActFault : STRUCT
     StartTime : DINT ;
     StartEdge : BOOL ;
    END_STRUCT ;
    DataTimeExtFault : STRUCT
     StartTime : DINT ;
     StartEdge : BOOL ;
    END_STRUCT ;
    DataTimeFeedback : STRUCT
     StartTime : DINT ;
     StartEdge : BOOL ;
    END_STRUCT ;
    DataTimeAutoAl : STRUCT
     StartTime : DINT ;
     StartEdge : BOOL ;
    END_STRUCT ;
    PCONF : STRUCT 	//// PCONF MOTOR1 - Instance 024
     Modeswitches : STRUCT
      M0_ConstantOut : BOOL ;	// Constant Output MST1 MST2 MSTO (1); Feedback depended Output Anst. (0)
      M1_AutoManLoc : BOOL ;	// AUTO/ MANUAL/ LOCAL (1); MANUAL/ LOCAL (0)
      M2_NoActFeedFault : BOOL ;	// No Action- and Non-Feedback fault(1),
      M3_NoStopIfFault : BOOL ;	// No Stop-Signal if Failure occurs (1)
      M4_RestrtAftBlack : BOOL ;	// Restart after Blackout (1)
      M5_ResetOSonly : BOOL ;	// Reset Alarm only with RESET from OS (1); RESET and START/STOP-Command (0)
      M6_CmdTimeDly : BOOL ;	// Command Time Delay aktiv (1)
      M7_Chg12viaStop : BOOL ;	// Change from 1->2 via STOP(1)
      M8_Chg21viaStop : BOOL ;	// Change from 2->1 via STOP(1)
      M9_StopIfAutoFail : BOOL ;	// NO AVAIL Direct Stop if Auto Failure (1)
      M10_LockBlockCmd : BOOL ;	// Lock blocksCommands
      sw11 : BOOL ;
      sw12 : BOOL ;
      sw13 : BOOL ;
      sw14 : BOOL ;
      sw15 : BOOL ;	//
     END_STRUCT ;
     DlyTCmd : TIME ;	// Setpoint Command time delay
     DlyTBlackout : TIME ;	// Setpoint blackout time delay
     DlyTExtFault : TIME ;	// Setpoint external fault delay
     DlyTFeedback : TIME ;	// Setpoint feedback fault delay
     DlyTActFault : TIME ;	// Setpoint Action Fault delay
     DlyTAutoAl : TIME ;	// Setpoint auto alarm delay
     DlyTRestart : TIME ;	// No AVAIL Setpoint restart after blackout delay
     DlyTChg12 : TIME ;	// Setpoint Waiting Delay 1->2
     DlyTChg21 : TIME ;	// Setpoint Waiting Delay 2->1
    END_STRUCT ;
   END_STRUCT ;
   MOTOR2_No025 : STRUCT
    System : WORD ;
    CmdOS : WORD ;
    MirrorCmdOS : WORD ;
    Test : WORD ;
    AlarmOS : WORD ;
    StatusOS : WORD ;
    SysStatusOS : WORD ;
    Status1 : WORD ;
    Status2 : WORD ;
    Status3 : BYTE ;
    InputEdges : BYTE ;
    AutoEdges : WORD ;
    DataTimeCmd : STRUCT
     StartTime : DINT ;
     StartEdge : BOOL ;
    END_STRUCT ;
    DataTimeChg12 : STRUCT
     StartTime : DINT ;
     StartEdge : BOOL ;
    END_STRUCT ;
    DataTimeChg21 : STRUCT
     StartTime : DINT ;
     StartEdge : BOOL ;
    END_STRUCT ;
    DataTimeBlackout : STRUCT
     StartTime : DINT ;
     StartEdge : BOOL ;
    END_STRUCT ;
    DataTimeActFault : STRUCT
     StartTime : DINT ;
     StartEdge : BOOL ;
    END_STRUCT ;
    DataTimeExtFault : STRUCT
     StartTime : DINT ;
     StartEdge : BOOL ;
    END_STRUCT ;
    DataTimeFeedback : STRUCT
     StartTime : DINT ;
     StartEdge : BOOL ;
    END_STRUCT ;
    DataTimeAutoAl : STRUCT
     StartTime : DINT ;
     StartEdge : BOOL ;
    END_STRUCT ;
    PCONF : STRUCT 	//// PCONF MOTOR1 - Instance 025
     Modeswitches : STRUCT
      M0_ConstantOut : BOOL ;	// Constant Output MST1 MST2 MSTO (1); Feedback depended Output Anst. (0)
      M1_AutoManLoc : BOOL ;	// AUTO/ MANUAL/ LOCAL (1); MANUAL/ LOCAL (0)
      M2_NoActFeedFault : BOOL ;	// No Action- and Non-Feedback fault(1),
      M3_NoStopIfFault : BOOL ;	// No Stop-Signal if Failure occurs (1)
      M4_RestrtAftBlack : BOOL ;	// Restart after Blackout (1)
      M5_ResetOSonly : BOOL ;	// Reset Alarm only with RESET from OS (1); RESET and START/STOP-Command (0)
      M6_CmdTimeDly : BOOL ;	// Command Time Delay aktiv (1)
      M7_Chg12viaStop : BOOL ;	// Change from 1->2 via STOP(1)
      M8_Chg21viaStop : BOOL ;	// Change from 2->1 via STOP(1)
      M9_StopIfAutoFail : BOOL ;	// NO AVAIL Direct Stop if Auto Failure (1)
      M10_LockBlockCmd : BOOL ;	// Lock blocksCommands
      sw11 : BOOL ;
      sw12 : BOOL ;
      sw13 : BOOL ;
      sw14 : BOOL ;
      sw15 : BOOL ;	//
     END_STRUCT ;
     DlyTCmd : TIME ;	// Setpoint Command time delay
     DlyTBlackout : TIME ;	// Setpoint blackout time delay
     DlyTExtFault : TIME ;	// Setpoint external fault delay
     DlyTFeedback : TIME ;	// Setpoint feedback fault delay
     DlyTActFault : TIME ;	// Setpoint Action Fault delay
     DlyTAutoAl : TIME ;	// Setpoint auto alarm delay
     DlyTRestart : TIME ;	// No AVAIL Setpoint restart after blackout delay
     DlyTChg12 : TIME ;	// Setpoint Waiting Delay 1->2
     DlyTChg21 : TIME ;	// Setpoint Waiting Delay 2->1
    END_STRUCT ;
   END_STRUCT ;
  END_STRUCT ;
BEGIN
   MOTOR2_No001.System := W#16#0;
   MOTOR2_No001.CmdOS := W#16#0;
   MOTOR2_No001.MirrorCmdOS := W#16#0;
   MOTOR2_No001.Test := W#16#0;
   MOTOR2_No001.AlarmOS := W#16#0;
   MOTOR2_No001.StatusOS := W#16#0;
   MOTOR2_No001.SysStatusOS := W#16#0;
   MOTOR2_No001.Status1 := W#16#0;
   MOTOR2_No001.Status2 := W#16#0;
   MOTOR2_No001.Status3 := B#16#0;
   MOTOR2_No001.InputEdges := B#16#0;
   MOTOR2_No001.AutoEdges := W#16#0;
   MOTOR2_No001.DataTimeCmd.StartTime := L#0;
   MOTOR2_No001.DataTimeCmd.StartEdge := FALSE;
   MOTOR2_No001.DataTimeChg12.StartTime := L#0;
   MOTOR2_No001.DataTimeChg12.StartEdge := FALSE;
   MOTOR2_No001.DataTimeChg21.StartTime := L#0;
   MOTOR2_No001.DataTimeChg21.StartEdge := FALSE;
   MOTOR2_No001.DataTimeBlackout.StartTime := L#0;
   MOTOR2_No001.DataTimeBlackout.StartEdge := FALSE;
   MOTOR2_No001.DataTimeActFault.StartTime := L#0;
   MOTOR2_No001.DataTimeActFault.StartEdge := FALSE;
   MOTOR2_No001.DataTimeExtFault.StartTime := L#0;
   MOTOR2_No001.DataTimeExtFault.StartEdge := FALSE;
   MOTOR2_No001.DataTimeFeedback.StartTime := L#0;
   MOTOR2_No001.DataTimeFeedback.StartEdge := FALSE;
   MOTOR2_No001.DataTimeAutoAl.StartTime := L#0;
   MOTOR2_No001.DataTimeAutoAl.StartEdge := FALSE;
   MOTOR2_No001.PCONF.Modeswitches.M0_ConstantOut := TRUE;
   MOTOR2_No001.PCONF.Modeswitches.M1_AutoManLoc := TRUE;
   MOTOR2_No001.PCONF.Modeswitches.M2_NoActFeedFault := FALSE;
   MOTOR2_No001.PCONF.Modeswitches.M3_NoStopIfFault := TRUE;
   MOTOR2_No001.PCONF.Modeswitches.M4_RestrtAftBlack := TRUE;
   MOTOR2_No001.PCONF.Modeswitches.M5_ResetOSonly := TRUE;
   MOTOR2_No001.PCONF.Modeswitches.M6_CmdTimeDly := FALSE;
   MOTOR2_No001.PCONF.Modeswitches.M7_Chg12viaStop := FALSE;
   MOTOR2_No001.PCONF.Modeswitches.M8_Chg21viaStop := FALSE;
   MOTOR2_No001.PCONF.Modeswitches.M9_StopIfAutoFail := FALSE;
   MOTOR2_No001.PCONF.Modeswitches.M10_LockBlockCmd := FALSE;
   MOTOR2_No001.PCONF.Modeswitches.sw11 := FALSE;
   MOTOR2_No001.PCONF.Modeswitches.sw12 := FALSE;
   MOTOR2_No001.PCONF.Modeswitches.sw13 := FALSE;
   MOTOR2_No001.PCONF.Modeswitches.sw14 := FALSE;
   MOTOR2_No001.PCONF.Modeswitches.sw15 := FALSE;
   MOTOR2_No001.PCONF.DlyTCmd := T#0MS;
   MOTOR2_No001.PCONF.DlyTBlackout := T#30S;
   MOTOR2_No001.PCONF.DlyTExtFault := T#2S;
   MOTOR2_No001.PCONF.DlyTFeedback := T#1S;
   MOTOR2_No001.PCONF.DlyTActFault := T#5S;
   MOTOR2_No001.PCONF.DlyTAutoAl := T#3S;
   MOTOR2_No001.PCONF.DlyTRestart := T#0MS;
   MOTOR2_No001.PCONF.DlyTChg12 := T#500MS;
   MOTOR2_No001.PCONF.DlyTChg21 := T#500MS;
   MOTOR2_No002.System := W#16#0;
   MOTOR2_No002.CmdOS := W#16#0;
   MOTOR2_No002.MirrorCmdOS := W#16#0;
   MOTOR2_No002.Test := W#16#0;
   MOTOR2_No002.AlarmOS := W#16#0;
   MOTOR2_No002.StatusOS := W#16#0;
   MOTOR2_No002.SysStatusOS := W#16#0;
   MOTOR2_No002.Status1 := W#16#0;
   MOTOR2_No002.Status2 := W#16#0;
   MOTOR2_No002.Status3 := B#16#0;
   MOTOR2_No002.InputEdges := B#16#0;
   MOTOR2_No002.AutoEdges := W#16#0;
   MOTOR2_No002.DataTimeCmd.StartTime := L#0;
   MOTOR2_No002.DataTimeCmd.StartEdge := FALSE;
   MOTOR2_No002.DataTimeChg12.StartTime := L#0;
   MOTOR2_No002.DataTimeChg12.StartEdge := FALSE;
   MOTOR2_No002.DataTimeChg21.StartTime := L#0;
   MOTOR2_No002.DataTimeChg21.StartEdge := FALSE;
   MOTOR2_No002.DataTimeBlackout.StartTime := L#0;
   MOTOR2_No002.DataTimeBlackout.StartEdge := FALSE;
   MOTOR2_No002.DataTimeActFault.StartTime := L#0;
   MOTOR2_No002.DataTimeActFault.StartEdge := FALSE;
   MOTOR2_No002.DataTimeExtFault.StartTime := L#0;
   MOTOR2_No002.DataTimeExtFault.StartEdge := FALSE;
   MOTOR2_No002.DataTimeFeedback.StartTime := L#0;
   MOTOR2_No002.DataTimeFeedback.StartEdge := FALSE;
   MOTOR2_No002.DataTimeAutoAl.StartTime := L#0;
   MOTOR2_No002.DataTimeAutoAl.StartEdge := FALSE;
   MOTOR2_No002.PCONF.Modeswitches.M0_ConstantOut := TRUE;
   MOTOR2_No002.PCONF.Modeswitches.M1_AutoManLoc := TRUE;
   MOTOR2_No002.PCONF.Modeswitches.M2_NoActFeedFault := FALSE;
   MOTOR2_No002.PCONF.Modeswitches.M3_NoStopIfFault := TRUE;
   MOTOR2_No002.PCONF.Modeswitches.M4_RestrtAftBlack := TRUE;
   MOTOR2_No002.PCONF.Modeswitches.M5_ResetOSonly := TRUE;
   MOTOR2_No002.PCONF.Modeswitches.M6_CmdTimeDly := FALSE;
   MOTOR2_No002.PCONF.Modeswitches.M7_Chg12viaStop := FALSE;
   MOTOR2_No002.PCONF.Modeswitches.M8_Chg21viaStop := FALSE;
   MOTOR2_No002.PCONF.Modeswitches.M9_StopIfAutoFail := FALSE;
   MOTOR2_No002.PCONF.Modeswitches.M10_LockBlockCmd := FALSE;
   MOTOR2_No002.PCONF.Modeswitches.sw11 := FALSE;
   MOTOR2_No002.PCONF.Modeswitches.sw12 := FALSE;
   MOTOR2_No002.PCONF.Modeswitches.sw13 := FALSE;
   MOTOR2_No002.PCONF.Modeswitches.sw14 := FALSE;
   MOTOR2_No002.PCONF.Modeswitches.sw15 := FALSE;
   MOTOR2_No002.PCONF.DlyTCmd := T#0MS;
   MOTOR2_No002.PCONF.DlyTBlackout := T#30S;
   MOTOR2_No002.PCONF.DlyTExtFault := T#2S;
   MOTOR2_No002.PCONF.DlyTFeedback := T#1S;
   MOTOR2_No002.PCONF.DlyTActFault := T#5S;
   MOTOR2_No002.PCONF.DlyTAutoAl := T#3S;
   MOTOR2_No002.PCONF.DlyTRestart := T#0MS;
   MOTOR2_No002.PCONF.DlyTChg12 := T#500MS;
   MOTOR2_No002.PCONF.DlyTChg21 := T#500MS;
   MOTOR2_No003.System := W#16#0;
   MOTOR2_No003.CmdOS := W#16#0;
   MOTOR2_No003.MirrorCmdOS := W#16#0;
   MOTOR2_No003.Test := W#16#0;
   MOTOR2_No003.AlarmOS := W#16#0;
   MOTOR2_No003.StatusOS := W#16#0;
   MOTOR2_No003.SysStatusOS := W#16#0;
   MOTOR2_No003.Status1 := W#16#0;
   MOTOR2_No003.Status2 := W#16#0;
   MOTOR2_No003.Status3 := B#16#0;
   MOTOR2_No003.InputEdges := B#16#0;
   MOTOR2_No003.AutoEdges := W#16#0;
   MOTOR2_No003.DataTimeCmd.StartTime := L#0;
   MOTOR2_No003.DataTimeCmd.StartEdge := FALSE;
   MOTOR2_No003.DataTimeChg12.StartTime := L#0;
   MOTOR2_No003.DataTimeChg12.StartEdge := FALSE;
   MOTOR2_No003.DataTimeChg21.StartTime := L#0;
   MOTOR2_No003.DataTimeChg21.StartEdge := FALSE;
   MOTOR2_No003.DataTimeBlackout.StartTime := L#0;
   MOTOR2_No003.DataTimeBlackout.StartEdge := FALSE;
   MOTOR2_No003.DataTimeActFault.StartTime := L#0;
   MOTOR2_No003.DataTimeActFault.StartEdge := FALSE;
   MOTOR2_No003.DataTimeExtFault.StartTime := L#0;
   MOTOR2_No003.DataTimeExtFault.StartEdge := FALSE;
   MOTOR2_No003.DataTimeFeedback.StartTime := L#0;
   MOTOR2_No003.DataTimeFeedback.StartEdge := FALSE;
   MOTOR2_No003.DataTimeAutoAl.StartTime := L#0;
   MOTOR2_No003.DataTimeAutoAl.StartEdge := FALSE;
   MOTOR2_No003.PCONF.Modeswitches.M0_ConstantOut := TRUE;
   MOTOR2_No003.PCONF.Modeswitches.M1_AutoManLoc := TRUE;
   MOTOR2_No003.PCONF.Modeswitches.M2_NoActFeedFault := FALSE;
   MOTOR2_No003.PCONF.Modeswitches.M3_NoStopIfFault := TRUE;
   MOTOR2_No003.PCONF.Modeswitches.M4_RestrtAftBlack := TRUE;
   MOTOR2_No003.PCONF.Modeswitches.M5_ResetOSonly := TRUE;
   MOTOR2_No003.PCONF.Modeswitches.M6_CmdTimeDly := FALSE;
   MOTOR2_No003.PCONF.Modeswitches.M7_Chg12viaStop := FALSE;
   MOTOR2_No003.PCONF.Modeswitches.M8_Chg21viaStop := FALSE;
   MOTOR2_No003.PCONF.Modeswitches.M9_StopIfAutoFail := FALSE;
   MOTOR2_No003.PCONF.Modeswitches.M10_LockBlockCmd := FALSE;
   MOTOR2_No003.PCONF.Modeswitches.sw11 := FALSE;
   MOTOR2_No003.PCONF.Modeswitches.sw12 := FALSE;
   MOTOR2_No003.PCONF.Modeswitches.sw13 := FALSE;
   MOTOR2_No003.PCONF.Modeswitches.sw14 := FALSE;
   MOTOR2_No003.PCONF.Modeswitches.sw15 := FALSE;
   MOTOR2_No003.PCONF.DlyTCmd := T#0MS;
   MOTOR2_No003.PCONF.DlyTBlackout := T#30S;
   MOTOR2_No003.PCONF.DlyTExtFault := T#2S;
   MOTOR2_No003.PCONF.DlyTFeedback := T#1S;
   MOTOR2_No003.PCONF.DlyTActFault := T#5S;
   MOTOR2_No003.PCONF.DlyTAutoAl := T#3S;
   MOTOR2_No003.PCONF.DlyTRestart := T#0MS;
   MOTOR2_No003.PCONF.DlyTChg12 := T#500MS;
   MOTOR2_No003.PCONF.DlyTChg21 := T#500MS;
   MOTOR2_No0004.System := W#16#0;
   MOTOR2_No0004.CmdOS := W#16#0;
   MOTOR2_No0004.MirrorCmdOS := W#16#0;
   MOTOR2_No0004.Test := W#16#0;
   MOTOR2_No0004.AlarmOS := W#16#0;
   MOTOR2_No0004.StatusOS := W#16#0;
   MOTOR2_No0004.SysStatusOS := W#16#0;
   MOTOR2_No0004.Status1 := W#16#0;
   MOTOR2_No0004.Status2 := W#16#0;
   MOTOR2_No0004.Status3 := B#16#0;
   MOTOR2_No0004.InputEdges := B#16#0;
   MOTOR2_No0004.AutoEdges := W#16#0;
   MOTOR2_No0004.DataTimeCmd.StartTime := L#0;
   MOTOR2_No0004.DataTimeCmd.StartEdge := FALSE;
   MOTOR2_No0004.DataTimeChg12.StartTime := L#0;
   MOTOR2_No0004.DataTimeChg12.StartEdge := FALSE;
   MOTOR2_No0004.DataTimeChg21.StartTime := L#0;
   MOTOR2_No0004.DataTimeChg21.StartEdge := FALSE;
   MOTOR2_No0004.DataTimeBlackout.StartTime := L#0;
   MOTOR2_No0004.DataTimeBlackout.StartEdge := FALSE;
   MOTOR2_No0004.DataTimeActFault.StartTime := L#0;
   MOTOR2_No0004.DataTimeActFault.StartEdge := FALSE;
   MOTOR2_No0004.DataTimeExtFault.StartTime := L#0;
   MOTOR2_No0004.DataTimeExtFault.StartEdge := FALSE;
   MOTOR2_No0004.DataTimeFeedback.StartTime := L#0;
   MOTOR2_No0004.DataTimeFeedback.StartEdge := FALSE;
   MOTOR2_No0004.DataTimeAutoAl.StartTime := L#0;
   MOTOR2_No0004.DataTimeAutoAl.StartEdge := FALSE;
   MOTOR2_No0004.PCONF.Modeswitches.M0_ConstantOut := FALSE;
   MOTOR2_No0004.PCONF.Modeswitches.M1_AutoManLoc := FALSE;
   MOTOR2_No0004.PCONF.Modeswitches.M2_NoActFeedFault := FALSE;
   MOTOR2_No0004.PCONF.Modeswitches.M3_NoStopIfFault := FALSE;
   MOTOR2_No0004.PCONF.Modeswitches.M4_RestrtAftBlack := FALSE;
   MOTOR2_No0004.PCONF.Modeswitches.M5_ResetOSonly := FALSE;
   MOTOR2_No0004.PCONF.Modeswitches.M6_CmdTimeDly := FALSE;
   MOTOR2_No0004.PCONF.Modeswitches.M7_Chg12viaStop := FALSE;
   MOTOR2_No0004.PCONF.Modeswitches.M8_Chg21viaStop := FALSE;
   MOTOR2_No0004.PCONF.Modeswitches.M9_StopIfAutoFail := FALSE;
   MOTOR2_No0004.PCONF.Modeswitches.M10_LockBlockCmd := FALSE;
   MOTOR2_No0004.PCONF.Modeswitches.sw11 := FALSE;
   MOTOR2_No0004.PCONF.Modeswitches.sw12 := FALSE;
   MOTOR2_No0004.PCONF.Modeswitches.sw13 := FALSE;
   MOTOR2_No0004.PCONF.Modeswitches.sw14 := FALSE;
   MOTOR2_No0004.PCONF.Modeswitches.sw15 := FALSE;
   MOTOR2_No0004.PCONF.DlyTCmd := T#0MS;
   MOTOR2_No0004.PCONF.DlyTBlackout := T#0MS;
   MOTOR2_No0004.PCONF.DlyTExtFault := T#0MS;
   MOTOR2_No0004.PCONF.DlyTFeedback := T#0MS;
   MOTOR2_No0004.PCONF.DlyTActFault := T#0MS;
   MOTOR2_No0004.PCONF.DlyTAutoAl := T#0MS;
   MOTOR2_No0004.PCONF.DlyTRestart := T#0MS;
   MOTOR2_No0004.PCONF.DlyTChg12 := T#0MS;
   MOTOR2_No0004.PCONF.DlyTChg21 := T#0MS;
   MOTOR2_No005.System := W#16#0;
   MOTOR2_No005.CmdOS := W#16#0;
   MOTOR2_No005.MirrorCmdOS := W#16#0;
   MOTOR2_No005.Test := W#16#0;
   MOTOR2_No005.AlarmOS := W#16#0;
   MOTOR2_No005.StatusOS := W#16#0;
   MOTOR2_No005.SysStatusOS := W#16#0;
   MOTOR2_No005.Status1 := W#16#0;
   MOTOR2_No005.Status2 := W#16#0;
   MOTOR2_No005.Status3 := B#16#0;
   MOTOR2_No005.InputEdges := B#16#0;
   MOTOR2_No005.AutoEdges := W#16#0;
   MOTOR2_No005.DataTimeCmd.StartTime := L#0;
   MOTOR2_No005.DataTimeCmd.StartEdge := FALSE;
   MOTOR2_No005.DataTimeChg12.StartTime := L#0;
   MOTOR2_No005.DataTimeChg12.StartEdge := FALSE;
   MOTOR2_No005.DataTimeChg21.StartTime := L#0;
   MOTOR2_No005.DataTimeChg21.StartEdge := FALSE;
   MOTOR2_No005.DataTimeBlackout.StartTime := L#0;
   MOTOR2_No005.DataTimeBlackout.StartEdge := FALSE;
   MOTOR2_No005.DataTimeActFault.StartTime := L#0;
   MOTOR2_No005.DataTimeActFault.StartEdge := FALSE;
   MOTOR2_No005.DataTimeExtFault.StartTime := L#0;
   MOTOR2_No005.DataTimeExtFault.StartEdge := FALSE;
   MOTOR2_No005.DataTimeFeedback.StartTime := L#0;
   MOTOR2_No005.DataTimeFeedback.StartEdge := FALSE;
   MOTOR2_No005.DataTimeAutoAl.StartTime := L#0;
   MOTOR2_No005.DataTimeAutoAl.StartEdge := FALSE;
   MOTOR2_No005.PCONF.Modeswitches.M0_ConstantOut := FALSE;
   MOTOR2_No005.PCONF.Modeswitches.M1_AutoManLoc := FALSE;
   MOTOR2_No005.PCONF.Modeswitches.M2_NoActFeedFault := FALSE;
   MOTOR2_No005.PCONF.Modeswitches.M3_NoStopIfFault := FALSE;
   MOTOR2_No005.PCONF.Modeswitches.M4_RestrtAftBlack := FALSE;
   MOTOR2_No005.PCONF.Modeswitches.M5_ResetOSonly := FALSE;
   MOTOR2_No005.PCONF.Modeswitches.M6_CmdTimeDly := FALSE;
   MOTOR2_No005.PCONF.Modeswitches.M7_Chg12viaStop := FALSE;
   MOTOR2_No005.PCONF.Modeswitches.M8_Chg21viaStop := FALSE;
   MOTOR2_No005.PCONF.Modeswitches.M9_StopIfAutoFail := FALSE;
   MOTOR2_No005.PCONF.Modeswitches.M10_LockBlockCmd := FALSE;
   MOTOR2_No005.PCONF.Modeswitches.sw11 := FALSE;
   MOTOR2_No005.PCONF.Modeswitches.sw12 := FALSE;
   MOTOR2_No005.PCONF.Modeswitches.sw13 := FALSE;
   MOTOR2_No005.PCONF.Modeswitches.sw14 := FALSE;
   MOTOR2_No005.PCONF.Modeswitches.sw15 := FALSE;
   MOTOR2_No005.PCONF.DlyTCmd := T#0MS;
   MOTOR2_No005.PCONF.DlyTBlackout := T#0MS;
   MOTOR2_No005.PCONF.DlyTExtFault := T#0MS;
   MOTOR2_No005.PCONF.DlyTFeedback := T#0MS;
   MOTOR2_No005.PCONF.DlyTActFault := T#0MS;
   MOTOR2_No005.PCONF.DlyTAutoAl := T#0MS;
   MOTOR2_No005.PCONF.DlyTRestart := T#0MS;
   MOTOR2_No005.PCONF.DlyTChg12 := T#0MS;
   MOTOR2_No005.PCONF.DlyTChg21 := T#0MS;
   MOTOR2_No006.System := W#16#0;
   MOTOR2_No006.CmdOS := W#16#0;
   MOTOR2_No006.MirrorCmdOS := W#16#0;
   MOTOR2_No006.Test := W#16#0;
   MOTOR2_No006.AlarmOS := W#16#0;
   MOTOR2_No006.StatusOS := W#16#0;
   MOTOR2_No006.SysStatusOS := W#16#0;
   MOTOR2_No006.Status1 := W#16#0;
   MOTOR2_No006.Status2 := W#16#0;
   MOTOR2_No006.Status3 := B#16#0;
   MOTOR2_No006.InputEdges := B#16#0;
   MOTOR2_No006.AutoEdges := W#16#0;
   MOTOR2_No006.DataTimeCmd.StartTime := L#0;
   MOTOR2_No006.DataTimeCmd.StartEdge := FALSE;
   MOTOR2_No006.DataTimeChg12.StartTime := L#0;
   MOTOR2_No006.DataTimeChg12.StartEdge := FALSE;
   MOTOR2_No006.DataTimeChg21.StartTime := L#0;
   MOTOR2_No006.DataTimeChg21.StartEdge := FALSE;
   MOTOR2_No006.DataTimeBlackout.StartTime := L#0;
   MOTOR2_No006.DataTimeBlackout.StartEdge := FALSE;
   MOTOR2_No006.DataTimeActFault.StartTime := L#0;
   MOTOR2_No006.DataTimeActFault.StartEdge := FALSE;
   MOTOR2_No006.DataTimeExtFault.StartTime := L#0;
   MOTOR2_No006.DataTimeExtFault.StartEdge := FALSE;
   MOTOR2_No006.DataTimeFeedback.StartTime := L#0;
   MOTOR2_No006.DataTimeFeedback.StartEdge := FALSE;
   MOTOR2_No006.DataTimeAutoAl.StartTime := L#0;
   MOTOR2_No006.DataTimeAutoAl.StartEdge := FALSE;
   MOTOR2_No006.PCONF.Modeswitches.M0_ConstantOut := FALSE;
   MOTOR2_No006.PCONF.Modeswitches.M1_AutoManLoc := FALSE;
   MOTOR2_No006.PCONF.Modeswitches.M2_NoActFeedFault := FALSE;
   MOTOR2_No006.PCONF.Modeswitches.M3_NoStopIfFault := FALSE;
   MOTOR2_No006.PCONF.Modeswitches.M4_RestrtAftBlack := FALSE;
   MOTOR2_No006.PCONF.Modeswitches.M5_ResetOSonly := FALSE;
   MOTOR2_No006.PCONF.Modeswitches.M6_CmdTimeDly := FALSE;
   MOTOR2_No006.PCONF.Modeswitches.M7_Chg12viaStop := FALSE;
   MOTOR2_No006.PCONF.Modeswitches.M8_Chg21viaStop := FALSE;
   MOTOR2_No006.PCONF.Modeswitches.M9_StopIfAutoFail := FALSE;
   MOTOR2_No006.PCONF.Modeswitches.M10_LockBlockCmd := FALSE;
   MOTOR2_No006.PCONF.Modeswitches.sw11 := FALSE;
   MOTOR2_No006.PCONF.Modeswitches.sw12 := FALSE;
   MOTOR2_No006.PCONF.Modeswitches.sw13 := FALSE;
   MOTOR2_No006.PCONF.Modeswitches.sw14 := FALSE;
   MOTOR2_No006.PCONF.Modeswitches.sw15 := FALSE;
   MOTOR2_No006.PCONF.DlyTCmd := T#0MS;
   MOTOR2_No006.PCONF.DlyTBlackout := T#0MS;
   MOTOR2_No006.PCONF.DlyTExtFault := T#0MS;
   MOTOR2_No006.PCONF.DlyTFeedback := T#0MS;
   MOTOR2_No006.PCONF.DlyTActFault := T#0MS;
   MOTOR2_No006.PCONF.DlyTAutoAl := T#0MS;
   MOTOR2_No006.PCONF.DlyTRestart := T#0MS;
   MOTOR2_No006.PCONF.DlyTChg12 := T#0MS;
   MOTOR2_No006.PCONF.DlyTChg21 := T#0MS;
   MOTOR2_No007.System := W#16#0;
   MOTOR2_No007.CmdOS := W#16#0;
   MOTOR2_No007.MirrorCmdOS := W#16#0;
   MOTOR2_No007.Test := W#16#0;
   MOTOR2_No007.AlarmOS := W#16#0;
   MOTOR2_No007.StatusOS := W#16#0;
   MOTOR2_No007.SysStatusOS := W#16#0;
   MOTOR2_No007.Status1 := W#16#0;
   MOTOR2_No007.Status2 := W#16#0;
   MOTOR2_No007.Status3 := B#16#0;
   MOTOR2_No007.InputEdges := B#16#0;
   MOTOR2_No007.AutoEdges := W#16#0;
   MOTOR2_No007.DataTimeCmd.StartTime := L#0;
   MOTOR2_No007.DataTimeCmd.StartEdge := FALSE;
   MOTOR2_No007.DataTimeChg12.StartTime := L#0;
   MOTOR2_No007.DataTimeChg12.StartEdge := FALSE;
   MOTOR2_No007.DataTimeChg21.StartTime := L#0;
   MOTOR2_No007.DataTimeChg21.StartEdge := FALSE;
   MOTOR2_No007.DataTimeBlackout.StartTime := L#0;
   MOTOR2_No007.DataTimeBlackout.StartEdge := FALSE;
   MOTOR2_No007.DataTimeActFault.StartTime := L#0;
   MOTOR2_No007.DataTimeActFault.StartEdge := FALSE;
   MOTOR2_No007.DataTimeExtFault.StartTime := L#0;
   MOTOR2_No007.DataTimeExtFault.StartEdge := FALSE;
   MOTOR2_No007.DataTimeFeedback.StartTime := L#0;
   MOTOR2_No007.DataTimeFeedback.StartEdge := FALSE;
   MOTOR2_No007.DataTimeAutoAl.StartTime := L#0;
   MOTOR2_No007.DataTimeAutoAl.StartEdge := FALSE;
   MOTOR2_No007.PCONF.Modeswitches.M0_ConstantOut := FALSE;
   MOTOR2_No007.PCONF.Modeswitches.M1_AutoManLoc := FALSE;
   MOTOR2_No007.PCONF.Modeswitches.M2_NoActFeedFault := FALSE;
   MOTOR2_No007.PCONF.Modeswitches.M3_NoStopIfFault := FALSE;
   MOTOR2_No007.PCONF.Modeswitches.M4_RestrtAftBlack := FALSE;
   MOTOR2_No007.PCONF.Modeswitches.M5_ResetOSonly := FALSE;
   MOTOR2_No007.PCONF.Modeswitches.M6_CmdTimeDly := FALSE;
   MOTOR2_No007.PCONF.Modeswitches.M7_Chg12viaStop := FALSE;
   MOTOR2_No007.PCONF.Modeswitches.M8_Chg21viaStop := FALSE;
   MOTOR2_No007.PCONF.Modeswitches.M9_StopIfAutoFail := FALSE;
   MOTOR2_No007.PCONF.Modeswitches.M10_LockBlockCmd := FALSE;
   MOTOR2_No007.PCONF.Modeswitches.sw11 := FALSE;
   MOTOR2_No007.PCONF.Modeswitches.sw12 := FALSE;
   MOTOR2_No007.PCONF.Modeswitches.sw13 := FALSE;
   MOTOR2_No007.PCONF.Modeswitches.sw14 := FALSE;
   MOTOR2_No007.PCONF.Modeswitches.sw15 := FALSE;
   MOTOR2_No007.PCONF.DlyTCmd := T#0MS;
   MOTOR2_No007.PCONF.DlyTBlackout := T#0MS;
   MOTOR2_No007.PCONF.DlyTExtFault := T#0MS;
   MOTOR2_No007.PCONF.DlyTFeedback := T#0MS;
   MOTOR2_No007.PCONF.DlyTActFault := T#0MS;
   MOTOR2_No007.PCONF.DlyTAutoAl := T#0MS;
   MOTOR2_No007.PCONF.DlyTRestart := T#0MS;
   MOTOR2_No007.PCONF.DlyTChg12 := T#0MS;
   MOTOR2_No007.PCONF.DlyTChg21 := T#0MS;
   MOTOR2_No008.System := W#16#0;
   MOTOR2_No008.CmdOS := W#16#0;
   MOTOR2_No008.MirrorCmdOS := W#16#0;
   MOTOR2_No008.Test := W#16#0;
   MOTOR2_No008.AlarmOS := W#16#0;
   MOTOR2_No008.StatusOS := W#16#0;
   MOTOR2_No008.SysStatusOS := W#16#0;
   MOTOR2_No008.Status1 := W#16#0;
   MOTOR2_No008.Status2 := W#16#0;
   MOTOR2_No008.Status3 := B#16#0;
   MOTOR2_No008.InputEdges := B#16#0;
   MOTOR2_No008.AutoEdges := W#16#0;
   MOTOR2_No008.DataTimeCmd.StartTime := L#0;
   MOTOR2_No008.DataTimeCmd.StartEdge := FALSE;
   MOTOR2_No008.DataTimeChg12.StartTime := L#0;
   MOTOR2_No008.DataTimeChg12.StartEdge := FALSE;
   MOTOR2_No008.DataTimeChg21.StartTime := L#0;
   MOTOR2_No008.DataTimeChg21.StartEdge := FALSE;
   MOTOR2_No008.DataTimeBlackout.StartTime := L#0;
   MOTOR2_No008.DataTimeBlackout.StartEdge := FALSE;
   MOTOR2_No008.DataTimeActFault.StartTime := L#0;
   MOTOR2_No008.DataTimeActFault.StartEdge := FALSE;
   MOTOR2_No008.DataTimeExtFault.StartTime := L#0;
   MOTOR2_No008.DataTimeExtFault.StartEdge := FALSE;
   MOTOR2_No008.DataTimeFeedback.StartTime := L#0;
   MOTOR2_No008.DataTimeFeedback.StartEdge := FALSE;
   MOTOR2_No008.DataTimeAutoAl.StartTime := L#0;
   MOTOR2_No008.DataTimeAutoAl.StartEdge := FALSE;
   MOTOR2_No008.PCONF.Modeswitches.M0_ConstantOut := FALSE;
   MOTOR2_No008.PCONF.Modeswitches.M1_AutoManLoc := FALSE;
   MOTOR2_No008.PCONF.Modeswitches.M2_NoActFeedFault := FALSE;
   MOTOR2_No008.PCONF.Modeswitches.M3_NoStopIfFault := FALSE;
   MOTOR2_No008.PCONF.Modeswitches.M4_RestrtAftBlack := FALSE;
   MOTOR2_No008.PCONF.Modeswitches.M5_ResetOSonly := FALSE;
   MOTOR2_No008.PCONF.Modeswitches.M6_CmdTimeDly := FALSE;
   MOTOR2_No008.PCONF.Modeswitches.M7_Chg12viaStop := FALSE;
   MOTOR2_No008.PCONF.Modeswitches.M8_Chg21viaStop := FALSE;
   MOTOR2_No008.PCONF.Modeswitches.M9_StopIfAutoFail := FALSE;
   MOTOR2_No008.PCONF.Modeswitches.M10_LockBlockCmd := FALSE;
   MOTOR2_No008.PCONF.Modeswitches.sw11 := FALSE;
   MOTOR2_No008.PCONF.Modeswitches.sw12 := FALSE;
   MOTOR2_No008.PCONF.Modeswitches.sw13 := FALSE;
   MOTOR2_No008.PCONF.Modeswitches.sw14 := FALSE;
   MOTOR2_No008.PCONF.Modeswitches.sw15 := FALSE;
   MOTOR2_No008.PCONF.DlyTCmd := T#0MS;
   MOTOR2_No008.PCONF.DlyTBlackout := T#0MS;
   MOTOR2_No008.PCONF.DlyTExtFault := T#0MS;
   MOTOR2_No008.PCONF.DlyTFeedback := T#0MS;
   MOTOR2_No008.PCONF.DlyTActFault := T#0MS;
   MOTOR2_No008.PCONF.DlyTAutoAl := T#0MS;
   MOTOR2_No008.PCONF.DlyTRestart := T#0MS;
   MOTOR2_No008.PCONF.DlyTChg12 := T#0MS;
   MOTOR2_No008.PCONF.DlyTChg21 := T#0MS;
   MOTOR2_No009.System := W#16#0;
   MOTOR2_No009.CmdOS := W#16#0;
   MOTOR2_No009.MirrorCmdOS := W#16#0;
   MOTOR2_No009.Test := W#16#0;
   MOTOR2_No009.AlarmOS := W#16#0;
   MOTOR2_No009.StatusOS := W#16#0;
   MOTOR2_No009.SysStatusOS := W#16#0;
   MOTOR2_No009.Status1 := W#16#0;
   MOTOR2_No009.Status2 := W#16#0;
   MOTOR2_No009.Status3 := B#16#0;
   MOTOR2_No009.InputEdges := B#16#0;
   MOTOR2_No009.AutoEdges := W#16#0;
   MOTOR2_No009.DataTimeCmd.StartTime := L#0;
   MOTOR2_No009.DataTimeCmd.StartEdge := FALSE;
   MOTOR2_No009.DataTimeChg12.StartTime := L#0;
   MOTOR2_No009.DataTimeChg12.StartEdge := FALSE;
   MOTOR2_No009.DataTimeChg21.StartTime := L#0;
   MOTOR2_No009.DataTimeChg21.StartEdge := FALSE;
   MOTOR2_No009.DataTimeBlackout.StartTime := L#0;
   MOTOR2_No009.DataTimeBlackout.StartEdge := FALSE;
   MOTOR2_No009.DataTimeActFault.StartTime := L#0;
   MOTOR2_No009.DataTimeActFault.StartEdge := FALSE;
   MOTOR2_No009.DataTimeExtFault.StartTime := L#0;
   MOTOR2_No009.DataTimeExtFault.StartEdge := FALSE;
   MOTOR2_No009.DataTimeFeedback.StartTime := L#0;
   MOTOR2_No009.DataTimeFeedback.StartEdge := FALSE;
   MOTOR2_No009.DataTimeAutoAl.StartTime := L#0;
   MOTOR2_No009.DataTimeAutoAl.StartEdge := FALSE;
   MOTOR2_No009.PCONF.Modeswitches.M0_ConstantOut := FALSE;
   MOTOR2_No009.PCONF.Modeswitches.M1_AutoManLoc := FALSE;
   MOTOR2_No009.PCONF.Modeswitches.M2_NoActFeedFault := FALSE;
   MOTOR2_No009.PCONF.Modeswitches.M3_NoStopIfFault := FALSE;
   MOTOR2_No009.PCONF.Modeswitches.M4_RestrtAftBlack := FALSE;
   MOTOR2_No009.PCONF.Modeswitches.M5_ResetOSonly := FALSE;
   MOTOR2_No009.PCONF.Modeswitches.M6_CmdTimeDly := FALSE;
   MOTOR2_No009.PCONF.Modeswitches.M7_Chg12viaStop := FALSE;
   MOTOR2_No009.PCONF.Modeswitches.M8_Chg21viaStop := FALSE;
   MOTOR2_No009.PCONF.Modeswitches.M9_StopIfAutoFail := FALSE;
   MOTOR2_No009.PCONF.Modeswitches.M10_LockBlockCmd := FALSE;
   MOTOR2_No009.PCONF.Modeswitches.sw11 := FALSE;
   MOTOR2_No009.PCONF.Modeswitches.sw12 := FALSE;
   MOTOR2_No009.PCONF.Modeswitches.sw13 := FALSE;
   MOTOR2_No009.PCONF.Modeswitches.sw14 := FALSE;
   MOTOR2_No009.PCONF.Modeswitches.sw15 := FALSE;
   MOTOR2_No009.PCONF.DlyTCmd := T#0MS;
   MOTOR2_No009.PCONF.DlyTBlackout := T#0MS;
   MOTOR2_No009.PCONF.DlyTExtFault := T#0MS;
   MOTOR2_No009.PCONF.DlyTFeedback := T#0MS;
   MOTOR2_No009.PCONF.DlyTActFault := T#0MS;
   MOTOR2_No009.PCONF.DlyTAutoAl := T#0MS;
   MOTOR2_No009.PCONF.DlyTRestart := T#0MS;
   MOTOR2_No009.PCONF.DlyTChg12 := T#0MS;
   MOTOR2_No009.PCONF.DlyTChg21 := T#0MS;
   MOTOR2_No010.System := W#16#0;
   MOTOR2_No010.CmdOS := W#16#0;
   MOTOR2_No010.MirrorCmdOS := W#16#0;
   MOTOR2_No010.Test := W#16#0;
   MOTOR2_No010.AlarmOS := W#16#0;
   MOTOR2_No010.StatusOS := W#16#0;
   MOTOR2_No010.SysStatusOS := W#16#0;
   MOTOR2_No010.Status1 := W#16#0;
   MOTOR2_No010.Status2 := W#16#0;
   MOTOR2_No010.Status3 := B#16#0;
   MOTOR2_No010.InputEdges := B#16#0;
   MOTOR2_No010.AutoEdges := W#16#0;
   MOTOR2_No010.DataTimeCmd.StartTime := L#0;
   MOTOR2_No010.DataTimeCmd.StartEdge := FALSE;
   MOTOR2_No010.DataTimeChg12.StartTime := L#0;
   MOTOR2_No010.DataTimeChg12.StartEdge := FALSE;
   MOTOR2_No010.DataTimeChg21.StartTime := L#0;
   MOTOR2_No010.DataTimeChg21.StartEdge := FALSE;
   MOTOR2_No010.DataTimeBlackout.StartTime := L#0;
   MOTOR2_No010.DataTimeBlackout.StartEdge := FALSE;
   MOTOR2_No010.DataTimeActFault.StartTime := L#0;
   MOTOR2_No010.DataTimeActFault.StartEdge := FALSE;
   MOTOR2_No010.DataTimeExtFault.StartTime := L#0;
   MOTOR2_No010.DataTimeExtFault.StartEdge := FALSE;
   MOTOR2_No010.DataTimeFeedback.StartTime := L#0;
   MOTOR2_No010.DataTimeFeedback.StartEdge := FALSE;
   MOTOR2_No010.DataTimeAutoAl.StartTime := L#0;
   MOTOR2_No010.DataTimeAutoAl.StartEdge := FALSE;
   MOTOR2_No010.PCONF.Modeswitches.M0_ConstantOut := FALSE;
   MOTOR2_No010.PCONF.Modeswitches.M1_AutoManLoc := FALSE;
   MOTOR2_No010.PCONF.Modeswitches.M2_NoActFeedFault := FALSE;
   MOTOR2_No010.PCONF.Modeswitches.M3_NoStopIfFault := FALSE;
   MOTOR2_No010.PCONF.Modeswitches.M4_RestrtAftBlack := FALSE;
   MOTOR2_No010.PCONF.Modeswitches.M5_ResetOSonly := FALSE;
   MOTOR2_No010.PCONF.Modeswitches.M6_CmdTimeDly := FALSE;
   MOTOR2_No010.PCONF.Modeswitches.M7_Chg12viaStop := FALSE;
   MOTOR2_No010.PCONF.Modeswitches.M8_Chg21viaStop := FALSE;
   MOTOR2_No010.PCONF.Modeswitches.M9_StopIfAutoFail := FALSE;
   MOTOR2_No010.PCONF.Modeswitches.M10_LockBlockCmd := FALSE;
   MOTOR2_No010.PCONF.Modeswitches.sw11 := FALSE;
   MOTOR2_No010.PCONF.Modeswitches.sw12 := FALSE;
   MOTOR2_No010.PCONF.Modeswitches.sw13 := FALSE;
   MOTOR2_No010.PCONF.Modeswitches.sw14 := FALSE;
   MOTOR2_No010.PCONF.Modeswitches.sw15 := FALSE;
   MOTOR2_No010.PCONF.DlyTCmd := T#0MS;
   MOTOR2_No010.PCONF.DlyTBlackout := T#0MS;
   MOTOR2_No010.PCONF.DlyTExtFault := T#0MS;
   MOTOR2_No010.PCONF.DlyTFeedback := T#0MS;
   MOTOR2_No010.PCONF.DlyTActFault := T#0MS;
   MOTOR2_No010.PCONF.DlyTAutoAl := T#0MS;
   MOTOR2_No010.PCONF.DlyTRestart := T#0MS;
   MOTOR2_No010.PCONF.DlyTChg12 := T#0MS;
   MOTOR2_No010.PCONF.DlyTChg21 := T#0MS;
   MOTOR2_No011.System := W#16#0;
   MOTOR2_No011.CmdOS := W#16#0;
   MOTOR2_No011.MirrorCmdOS := W#16#0;
   MOTOR2_No011.Test := W#16#0;
   MOTOR2_No011.AlarmOS := W#16#0;
   MOTOR2_No011.StatusOS := W#16#0;
   MOTOR2_No011.SysStatusOS := W#16#0;
   MOTOR2_No011.Status1 := W#16#0;
   MOTOR2_No011.Status2 := W#16#0;
   MOTOR2_No011.Status3 := B#16#0;
   MOTOR2_No011.InputEdges := B#16#0;
   MOTOR2_No011.AutoEdges := W#16#0;
   MOTOR2_No011.DataTimeCmd.StartTime := L#0;
   MOTOR2_No011.DataTimeCmd.StartEdge := FALSE;
   MOTOR2_No011.DataTimeChg12.StartTime := L#0;
   MOTOR2_No011.DataTimeChg12.StartEdge := FALSE;
   MOTOR2_No011.DataTimeChg21.StartTime := L#0;
   MOTOR2_No011.DataTimeChg21.StartEdge := FALSE;
   MOTOR2_No011.DataTimeBlackout.StartTime := L#0;
   MOTOR2_No011.DataTimeBlackout.StartEdge := FALSE;
   MOTOR2_No011.DataTimeActFault.StartTime := L#0;
   MOTOR2_No011.DataTimeActFault.StartEdge := FALSE;
   MOTOR2_No011.DataTimeExtFault.StartTime := L#0;
   MOTOR2_No011.DataTimeExtFault.StartEdge := FALSE;
   MOTOR2_No011.DataTimeFeedback.StartTime := L#0;
   MOTOR2_No011.DataTimeFeedback.StartEdge := FALSE;
   MOTOR2_No011.DataTimeAutoAl.StartTime := L#0;
   MOTOR2_No011.DataTimeAutoAl.StartEdge := FALSE;
   MOTOR2_No011.PCONF.Modeswitches.M0_ConstantOut := FALSE;
   MOTOR2_No011.PCONF.Modeswitches.M1_AutoManLoc := FALSE;
   MOTOR2_No011.PCONF.Modeswitches.M2_NoActFeedFault := FALSE;
   MOTOR2_No011.PCONF.Modeswitches.M3_NoStopIfFault := FALSE;
   MOTOR2_No011.PCONF.Modeswitches.M4_RestrtAftBlack := FALSE;
   MOTOR2_No011.PCONF.Modeswitches.M5_ResetOSonly := FALSE;
   MOTOR2_No011.PCONF.Modeswitches.M6_CmdTimeDly := FALSE;
   MOTOR2_No011.PCONF.Modeswitches.M7_Chg12viaStop := FALSE;
   MOTOR2_No011.PCONF.Modeswitches.M8_Chg21viaStop := FALSE;
   MOTOR2_No011.PCONF.Modeswitches.M9_StopIfAutoFail := FALSE;
   MOTOR2_No011.PCONF.Modeswitches.M10_LockBlockCmd := FALSE;
   MOTOR2_No011.PCONF.Modeswitches.sw11 := FALSE;
   MOTOR2_No011.PCONF.Modeswitches.sw12 := FALSE;
   MOTOR2_No011.PCONF.Modeswitches.sw13 := FALSE;
   MOTOR2_No011.PCONF.Modeswitches.sw14 := FALSE;
   MOTOR2_No011.PCONF.Modeswitches.sw15 := FALSE;
   MOTOR2_No011.PCONF.DlyTCmd := T#0MS;
   MOTOR2_No011.PCONF.DlyTBlackout := T#0MS;
   MOTOR2_No011.PCONF.DlyTExtFault := T#0MS;
   MOTOR2_No011.PCONF.DlyTFeedback := T#0MS;
   MOTOR2_No011.PCONF.DlyTActFault := T#0MS;
   MOTOR2_No011.PCONF.DlyTAutoAl := T#0MS;
   MOTOR2_No011.PCONF.DlyTRestart := T#0MS;
   MOTOR2_No011.PCONF.DlyTChg12 := T#0MS;
   MOTOR2_No011.PCONF.DlyTChg21 := T#0MS;
   MOTOR2_No012.System := W#16#0;
   MOTOR2_No012.CmdOS := W#16#0;
   MOTOR2_No012.MirrorCmdOS := W#16#0;
   MOTOR2_No012.Test := W#16#0;
   MOTOR2_No012.AlarmOS := W#16#0;
   MOTOR2_No012.StatusOS := W#16#0;
   MOTOR2_No012.SysStatusOS := W#16#0;
   MOTOR2_No012.Status1 := W#16#0;
   MOTOR2_No012.Status2 := W#16#0;
   MOTOR2_No012.Status3 := B#16#0;
   MOTOR2_No012.InputEdges := B#16#0;
   MOTOR2_No012.AutoEdges := W#16#0;
   MOTOR2_No012.DataTimeCmd.StartTime := L#0;
   MOTOR2_No012.DataTimeCmd.StartEdge := FALSE;
   MOTOR2_No012.DataTimeChg12.StartTime := L#0;
   MOTOR2_No012.DataTimeChg12.StartEdge := FALSE;
   MOTOR2_No012.DataTimeChg21.StartTime := L#0;
   MOTOR2_No012.DataTimeChg21.StartEdge := FALSE;
   MOTOR2_No012.DataTimeBlackout.StartTime := L#0;
   MOTOR2_No012.DataTimeBlackout.StartEdge := FALSE;
   MOTOR2_No012.DataTimeActFault.StartTime := L#0;
   MOTOR2_No012.DataTimeActFault.StartEdge := FALSE;
   MOTOR2_No012.DataTimeExtFault.StartTime := L#0;
   MOTOR2_No012.DataTimeExtFault.StartEdge := FALSE;
   MOTOR2_No012.DataTimeFeedback.StartTime := L#0;
   MOTOR2_No012.DataTimeFeedback.StartEdge := FALSE;
   MOTOR2_No012.DataTimeAutoAl.StartTime := L#0;
   MOTOR2_No012.DataTimeAutoAl.StartEdge := FALSE;
   MOTOR2_No012.PCONF.Modeswitches.M0_ConstantOut := FALSE;
   MOTOR2_No012.PCONF.Modeswitches.M1_AutoManLoc := FALSE;
   MOTOR2_No012.PCONF.Modeswitches.M2_NoActFeedFault := FALSE;
   MOTOR2_No012.PCONF.Modeswitches.M3_NoStopIfFault := FALSE;
   MOTOR2_No012.PCONF.Modeswitches.M4_RestrtAftBlack := FALSE;
   MOTOR2_No012.PCONF.Modeswitches.M5_ResetOSonly := FALSE;
   MOTOR2_No012.PCONF.Modeswitches.M6_CmdTimeDly := FALSE;
   MOTOR2_No012.PCONF.Modeswitches.M7_Chg12viaStop := FALSE;
   MOTOR2_No012.PCONF.Modeswitches.M8_Chg21viaStop := FALSE;
   MOTOR2_No012.PCONF.Modeswitches.M9_StopIfAutoFail := FALSE;
   MOTOR2_No012.PCONF.Modeswitches.M10_LockBlockCmd := FALSE;
   MOTOR2_No012.PCONF.Modeswitches.sw11 := FALSE;
   MOTOR2_No012.PCONF.Modeswitches.sw12 := FALSE;
   MOTOR2_No012.PCONF.Modeswitches.sw13 := FALSE;
   MOTOR2_No012.PCONF.Modeswitches.sw14 := FALSE;
   MOTOR2_No012.PCONF.Modeswitches.sw15 := FALSE;
   MOTOR2_No012.PCONF.DlyTCmd := T#0MS;
   MOTOR2_No012.PCONF.DlyTBlackout := T#0MS;
   MOTOR2_No012.PCONF.DlyTExtFault := T#0MS;
   MOTOR2_No012.PCONF.DlyTFeedback := T#0MS;
   MOTOR2_No012.PCONF.DlyTActFault := T#0MS;
   MOTOR2_No012.PCONF.DlyTAutoAl := T#0MS;
   MOTOR2_No012.PCONF.DlyTRestart := T#0MS;
   MOTOR2_No012.PCONF.DlyTChg12 := T#0MS;
   MOTOR2_No012.PCONF.DlyTChg21 := T#0MS;
   MOTOR2_No013.System := W#16#0;
   MOTOR2_No013.CmdOS := W#16#0;
   MOTOR2_No013.MirrorCmdOS := W#16#0;
   MOTOR2_No013.Test := W#16#0;
   MOTOR2_No013.AlarmOS := W#16#0;
   MOTOR2_No013.StatusOS := W#16#0;
   MOTOR2_No013.SysStatusOS := W#16#0;
   MOTOR2_No013.Status1 := W#16#0;
   MOTOR2_No013.Status2 := W#16#0;
   MOTOR2_No013.Status3 := B#16#0;
   MOTOR2_No013.InputEdges := B#16#0;
   MOTOR2_No013.AutoEdges := W#16#0;
   MOTOR2_No013.DataTimeCmd.StartTime := L#0;
   MOTOR2_No013.DataTimeCmd.StartEdge := FALSE;
   MOTOR2_No013.DataTimeChg12.StartTime := L#0;
   MOTOR2_No013.DataTimeChg12.StartEdge := FALSE;
   MOTOR2_No013.DataTimeChg21.StartTime := L#0;
   MOTOR2_No013.DataTimeChg21.StartEdge := FALSE;
   MOTOR2_No013.DataTimeBlackout.StartTime := L#0;
   MOTOR2_No013.DataTimeBlackout.StartEdge := FALSE;
   MOTOR2_No013.DataTimeActFault.StartTime := L#0;
   MOTOR2_No013.DataTimeActFault.StartEdge := FALSE;
   MOTOR2_No013.DataTimeExtFault.StartTime := L#0;
   MOTOR2_No013.DataTimeExtFault.StartEdge := FALSE;
   MOTOR2_No013.DataTimeFeedback.StartTime := L#0;
   MOTOR2_No013.DataTimeFeedback.StartEdge := FALSE;
   MOTOR2_No013.DataTimeAutoAl.StartTime := L#0;
   MOTOR2_No013.DataTimeAutoAl.StartEdge := FALSE;
   MOTOR2_No013.PCONF.Modeswitches.M0_ConstantOut := FALSE;
   MOTOR2_No013.PCONF.Modeswitches.M1_AutoManLoc := FALSE;
   MOTOR2_No013.PCONF.Modeswitches.M2_NoActFeedFault := FALSE;
   MOTOR2_No013.PCONF.Modeswitches.M3_NoStopIfFault := FALSE;
   MOTOR2_No013.PCONF.Modeswitches.M4_RestrtAftBlack := FALSE;
   MOTOR2_No013.PCONF.Modeswitches.M5_ResetOSonly := FALSE;
   MOTOR2_No013.PCONF.Modeswitches.M6_CmdTimeDly := FALSE;
   MOTOR2_No013.PCONF.Modeswitches.M7_Chg12viaStop := FALSE;
   MOTOR2_No013.PCONF.Modeswitches.M8_Chg21viaStop := FALSE;
   MOTOR2_No013.PCONF.Modeswitches.M9_StopIfAutoFail := FALSE;
   MOTOR2_No013.PCONF.Modeswitches.M10_LockBlockCmd := FALSE;
   MOTOR2_No013.PCONF.Modeswitches.sw11 := FALSE;
   MOTOR2_No013.PCONF.Modeswitches.sw12 := FALSE;
   MOTOR2_No013.PCONF.Modeswitches.sw13 := FALSE;
   MOTOR2_No013.PCONF.Modeswitches.sw14 := FALSE;
   MOTOR2_No013.PCONF.Modeswitches.sw15 := FALSE;
   MOTOR2_No013.PCONF.DlyTCmd := T#0MS;
   MOTOR2_No013.PCONF.DlyTBlackout := T#0MS;
   MOTOR2_No013.PCONF.DlyTExtFault := T#0MS;
   MOTOR2_No013.PCONF.DlyTFeedback := T#0MS;
   MOTOR2_No013.PCONF.DlyTActFault := T#0MS;
   MOTOR2_No013.PCONF.DlyTAutoAl := T#0MS;
   MOTOR2_No013.PCONF.DlyTRestart := T#0MS;
   MOTOR2_No013.PCONF.DlyTChg12 := T#0MS;
   MOTOR2_No013.PCONF.DlyTChg21 := T#0MS;
   MOTOR2_No014.System := W#16#0;
   MOTOR2_No014.CmdOS := W#16#0;
   MOTOR2_No014.MirrorCmdOS := W#16#0;
   MOTOR2_No014.Test := W#16#0;
   MOTOR2_No014.AlarmOS := W#16#0;
   MOTOR2_No014.StatusOS := W#16#0;
   MOTOR2_No014.SysStatusOS := W#16#0;
   MOTOR2_No014.Status1 := W#16#0;
   MOTOR2_No014.Status2 := W#16#0;
   MOTOR2_No014.Status3 := B#16#0;
   MOTOR2_No014.InputEdges := B#16#0;
   MOTOR2_No014.AutoEdges := W#16#0;
   MOTOR2_No014.DataTimeCmd.StartTime := L#0;
   MOTOR2_No014.DataTimeCmd.StartEdge := FALSE;
   MOTOR2_No014.DataTimeChg12.StartTime := L#0;
   MOTOR2_No014.DataTimeChg12.StartEdge := FALSE;
   MOTOR2_No014.DataTimeChg21.StartTime := L#0;
   MOTOR2_No014.DataTimeChg21.StartEdge := FALSE;
   MOTOR2_No014.DataTimeBlackout.StartTime := L#0;
   MOTOR2_No014.DataTimeBlackout.StartEdge := FALSE;
   MOTOR2_No014.DataTimeActFault.StartTime := L#0;
   MOTOR2_No014.DataTimeActFault.StartEdge := FALSE;
   MOTOR2_No014.DataTimeExtFault.StartTime := L#0;
   MOTOR2_No014.DataTimeExtFault.StartEdge := FALSE;
   MOTOR2_No014.DataTimeFeedback.StartTime := L#0;
   MOTOR2_No014.DataTimeFeedback.StartEdge := FALSE;
   MOTOR2_No014.DataTimeAutoAl.StartTime := L#0;
   MOTOR2_No014.DataTimeAutoAl.StartEdge := FALSE;
   MOTOR2_No014.PCONF.Modeswitches.M0_ConstantOut := FALSE;
   MOTOR2_No014.PCONF.Modeswitches.M1_AutoManLoc := FALSE;
   MOTOR2_No014.PCONF.Modeswitches.M2_NoActFeedFault := FALSE;
   MOTOR2_No014.PCONF.Modeswitches.M3_NoStopIfFault := FALSE;
   MOTOR2_No014.PCONF.Modeswitches.M4_RestrtAftBlack := FALSE;
   MOTOR2_No014.PCONF.Modeswitches.M5_ResetOSonly := FALSE;
   MOTOR2_No014.PCONF.Modeswitches.M6_CmdTimeDly := FALSE;
   MOTOR2_No014.PCONF.Modeswitches.M7_Chg12viaStop := FALSE;
   MOTOR2_No014.PCONF.Modeswitches.M8_Chg21viaStop := FALSE;
   MOTOR2_No014.PCONF.Modeswitches.M9_StopIfAutoFail := FALSE;
   MOTOR2_No014.PCONF.Modeswitches.M10_LockBlockCmd := FALSE;
   MOTOR2_No014.PCONF.Modeswitches.sw11 := FALSE;
   MOTOR2_No014.PCONF.Modeswitches.sw12 := FALSE;
   MOTOR2_No014.PCONF.Modeswitches.sw13 := FALSE;
   MOTOR2_No014.PCONF.Modeswitches.sw14 := FALSE;
   MOTOR2_No014.PCONF.Modeswitches.sw15 := FALSE;
   MOTOR2_No014.PCONF.DlyTCmd := T#0MS;
   MOTOR2_No014.PCONF.DlyTBlackout := T#0MS;
   MOTOR2_No014.PCONF.DlyTExtFault := T#0MS;
   MOTOR2_No014.PCONF.DlyTFeedback := T#0MS;
   MOTOR2_No014.PCONF.DlyTActFault := T#0MS;
   MOTOR2_No014.PCONF.DlyTAutoAl := T#0MS;
   MOTOR2_No014.PCONF.DlyTRestart := T#0MS;
   MOTOR2_No014.PCONF.DlyTChg12 := T#0MS;
   MOTOR2_No014.PCONF.DlyTChg21 := T#0MS;
   MOTOR2_No015.System := W#16#0;
   MOTOR2_No015.CmdOS := W#16#0;
   MOTOR2_No015.MirrorCmdOS := W#16#0;
   MOTOR2_No015.Test := W#16#0;
   MOTOR2_No015.AlarmOS := W#16#0;
   MOTOR2_No015.StatusOS := W#16#0;
   MOTOR2_No015.SysStatusOS := W#16#0;
   MOTOR2_No015.Status1 := W#16#0;
   MOTOR2_No015.Status2 := W#16#0;
   MOTOR2_No015.Status3 := B#16#0;
   MOTOR2_No015.InputEdges := B#16#0;
   MOTOR2_No015.AutoEdges := W#16#0;
   MOTOR2_No015.DataTimeCmd.StartTime := L#0;
   MOTOR2_No015.DataTimeCmd.StartEdge := FALSE;
   MOTOR2_No015.DataTimeChg12.StartTime := L#0;
   MOTOR2_No015.DataTimeChg12.StartEdge := FALSE;
   MOTOR2_No015.DataTimeChg21.StartTime := L#0;
   MOTOR2_No015.DataTimeChg21.StartEdge := FALSE;
   MOTOR2_No015.DataTimeBlackout.StartTime := L#0;
   MOTOR2_No015.DataTimeBlackout.StartEdge := FALSE;
   MOTOR2_No015.DataTimeActFault.StartTime := L#0;
   MOTOR2_No015.DataTimeActFault.StartEdge := FALSE;
   MOTOR2_No015.DataTimeExtFault.StartTime := L#0;
   MOTOR2_No015.DataTimeExtFault.StartEdge := FALSE;
   MOTOR2_No015.DataTimeFeedback.StartTime := L#0;
   MOTOR2_No015.DataTimeFeedback.StartEdge := FALSE;
   MOTOR2_No015.DataTimeAutoAl.StartTime := L#0;
   MOTOR2_No015.DataTimeAutoAl.StartEdge := FALSE;
   MOTOR2_No015.PCONF.Modeswitches.M0_ConstantOut := FALSE;
   MOTOR2_No015.PCONF.Modeswitches.M1_AutoManLoc := FALSE;
   MOTOR2_No015.PCONF.Modeswitches.M2_NoActFeedFault := FALSE;
   MOTOR2_No015.PCONF.Modeswitches.M3_NoStopIfFault := FALSE;
   MOTOR2_No015.PCONF.Modeswitches.M4_RestrtAftBlack := FALSE;
   MOTOR2_No015.PCONF.Modeswitches.M5_ResetOSonly := FALSE;
   MOTOR2_No015.PCONF.Modeswitches.M6_CmdTimeDly := FALSE;
   MOTOR2_No015.PCONF.Modeswitches.M7_Chg12viaStop := FALSE;
   MOTOR2_No015.PCONF.Modeswitches.M8_Chg21viaStop := FALSE;
   MOTOR2_No015.PCONF.Modeswitches.M9_StopIfAutoFail := FALSE;
   MOTOR2_No015.PCONF.Modeswitches.M10_LockBlockCmd := FALSE;
   MOTOR2_No015.PCONF.Modeswitches.sw11 := FALSE;
   MOTOR2_No015.PCONF.Modeswitches.sw12 := FALSE;
   MOTOR2_No015.PCONF.Modeswitches.sw13 := FALSE;
   MOTOR2_No015.PCONF.Modeswitches.sw14 := FALSE;
   MOTOR2_No015.PCONF.Modeswitches.sw15 := FALSE;
   MOTOR2_No015.PCONF.DlyTCmd := T#0MS;
   MOTOR2_No015.PCONF.DlyTBlackout := T#0MS;
   MOTOR2_No015.PCONF.DlyTExtFault := T#0MS;
   MOTOR2_No015.PCONF.DlyTFeedback := T#0MS;
   MOTOR2_No015.PCONF.DlyTActFault := T#0MS;
   MOTOR2_No015.PCONF.DlyTAutoAl := T#0MS;
   MOTOR2_No015.PCONF.DlyTRestart := T#0MS;
   MOTOR2_No015.PCONF.DlyTChg12 := T#0MS;
   MOTOR2_No015.PCONF.DlyTChg21 := T#0MS;
   MOTOR2_No016.System := W#16#0;
   MOTOR2_No016.CmdOS := W#16#0;
   MOTOR2_No016.MirrorCmdOS := W#16#0;
   MOTOR2_No016.Test := W#16#0;
   MOTOR2_No016.AlarmOS := W#16#0;
   MOTOR2_No016.StatusOS := W#16#0;
   MOTOR2_No016.SysStatusOS := W#16#0;
   MOTOR2_No016.Status1 := W#16#0;
   MOTOR2_No016.Status2 := W#16#0;
   MOTOR2_No016.Status3 := B#16#0;
   MOTOR2_No016.InputEdges := B#16#0;
   MOTOR2_No016.AutoEdges := W#16#0;
   MOTOR2_No016.DataTimeCmd.StartTime := L#0;
   MOTOR2_No016.DataTimeCmd.StartEdge := FALSE;
   MOTOR2_No016.DataTimeChg12.StartTime := L#0;
   MOTOR2_No016.DataTimeChg12.StartEdge := FALSE;
   MOTOR2_No016.DataTimeChg21.StartTime := L#0;
   MOTOR2_No016.DataTimeChg21.StartEdge := FALSE;
   MOTOR2_No016.DataTimeBlackout.StartTime := L#0;
   MOTOR2_No016.DataTimeBlackout.StartEdge := FALSE;
   MOTOR2_No016.DataTimeActFault.StartTime := L#0;
   MOTOR2_No016.DataTimeActFault.StartEdge := FALSE;
   MOTOR2_No016.DataTimeExtFault.StartTime := L#0;
   MOTOR2_No016.DataTimeExtFault.StartEdge := FALSE;
   MOTOR2_No016.DataTimeFeedback.StartTime := L#0;
   MOTOR2_No016.DataTimeFeedback.StartEdge := FALSE;
   MOTOR2_No016.DataTimeAutoAl.StartTime := L#0;
   MOTOR2_No016.DataTimeAutoAl.StartEdge := FALSE;
   MOTOR2_No016.PCONF.Modeswitches.M0_ConstantOut := FALSE;
   MOTOR2_No016.PCONF.Modeswitches.M1_AutoManLoc := FALSE;
   MOTOR2_No016.PCONF.Modeswitches.M2_NoActFeedFault := FALSE;
   MOTOR2_No016.PCONF.Modeswitches.M3_NoStopIfFault := FALSE;
   MOTOR2_No016.PCONF.Modeswitches.M4_RestrtAftBlack := FALSE;
   MOTOR2_No016.PCONF.Modeswitches.M5_ResetOSonly := FALSE;
   MOTOR2_No016.PCONF.Modeswitches.M6_CmdTimeDly := FALSE;
   MOTOR2_No016.PCONF.Modeswitches.M7_Chg12viaStop := FALSE;
   MOTOR2_No016.PCONF.Modeswitches.M8_Chg21viaStop := FALSE;
   MOTOR2_No016.PCONF.Modeswitches.M9_StopIfAutoFail := FALSE;
   MOTOR2_No016.PCONF.Modeswitches.M10_LockBlockCmd := FALSE;
   MOTOR2_No016.PCONF.Modeswitches.sw11 := FALSE;
   MOTOR2_No016.PCONF.Modeswitches.sw12 := FALSE;
   MOTOR2_No016.PCONF.Modeswitches.sw13 := FALSE;
   MOTOR2_No016.PCONF.Modeswitches.sw14 := FALSE;
   MOTOR2_No016.PCONF.Modeswitches.sw15 := FALSE;
   MOTOR2_No016.PCONF.DlyTCmd := T#0MS;
   MOTOR2_No016.PCONF.DlyTBlackout := T#0MS;
   MOTOR2_No016.PCONF.DlyTExtFault := T#0MS;
   MOTOR2_No016.PCONF.DlyTFeedback := T#0MS;
   MOTOR2_No016.PCONF.DlyTActFault := T#0MS;
   MOTOR2_No016.PCONF.DlyTAutoAl := T#0MS;
   MOTOR2_No016.PCONF.DlyTRestart := T#0MS;
   MOTOR2_No016.PCONF.DlyTChg12 := T#0MS;
   MOTOR2_No016.PCONF.DlyTChg21 := T#0MS;
   MOTOR2_No017.System := W#16#0;
   MOTOR2_No017.CmdOS := W#16#0;
   MOTOR2_No017.MirrorCmdOS := W#16#0;
   MOTOR2_No017.Test := W#16#0;
   MOTOR2_No017.AlarmOS := W#16#0;
   MOTOR2_No017.StatusOS := W#16#0;
   MOTOR2_No017.SysStatusOS := W#16#0;
   MOTOR2_No017.Status1 := W#16#0;
   MOTOR2_No017.Status2 := W#16#0;
   MOTOR2_No017.Status3 := B#16#0;
   MOTOR2_No017.InputEdges := B#16#0;
   MOTOR2_No017.AutoEdges := W#16#0;
   MOTOR2_No017.DataTimeCmd.StartTime := L#0;
   MOTOR2_No017.DataTimeCmd.StartEdge := FALSE;
   MOTOR2_No017.DataTimeChg12.StartTime := L#0;
   MOTOR2_No017.DataTimeChg12.StartEdge := FALSE;
   MOTOR2_No017.DataTimeChg21.StartTime := L#0;
   MOTOR2_No017.DataTimeChg21.StartEdge := FALSE;
   MOTOR2_No017.DataTimeBlackout.StartTime := L#0;
   MOTOR2_No017.DataTimeBlackout.StartEdge := FALSE;
   MOTOR2_No017.DataTimeActFault.StartTime := L#0;
   MOTOR2_No017.DataTimeActFault.StartEdge := FALSE;
   MOTOR2_No017.DataTimeExtFault.StartTime := L#0;
   MOTOR2_No017.DataTimeExtFault.StartEdge := FALSE;
   MOTOR2_No017.DataTimeFeedback.StartTime := L#0;
   MOTOR2_No017.DataTimeFeedback.StartEdge := FALSE;
   MOTOR2_No017.DataTimeAutoAl.StartTime := L#0;
   MOTOR2_No017.DataTimeAutoAl.StartEdge := FALSE;
   MOTOR2_No017.PCONF.Modeswitches.M0_ConstantOut := FALSE;
   MOTOR2_No017.PCONF.Modeswitches.M1_AutoManLoc := FALSE;
   MOTOR2_No017.PCONF.Modeswitches.M2_NoActFeedFault := FALSE;
   MOTOR2_No017.PCONF.Modeswitches.M3_NoStopIfFault := FALSE;
   MOTOR2_No017.PCONF.Modeswitches.M4_RestrtAftBlack := FALSE;
   MOTOR2_No017.PCONF.Modeswitches.M5_ResetOSonly := FALSE;
   MOTOR2_No017.PCONF.Modeswitches.M6_CmdTimeDly := FALSE;
   MOTOR2_No017.PCONF.Modeswitches.M7_Chg12viaStop := FALSE;
   MOTOR2_No017.PCONF.Modeswitches.M8_Chg21viaStop := FALSE;
   MOTOR2_No017.PCONF.Modeswitches.M9_StopIfAutoFail := FALSE;
   MOTOR2_No017.PCONF.Modeswitches.M10_LockBlockCmd := FALSE;
   MOTOR2_No017.PCONF.Modeswitches.sw11 := FALSE;
   MOTOR2_No017.PCONF.Modeswitches.sw12 := FALSE;
   MOTOR2_No017.PCONF.Modeswitches.sw13 := FALSE;
   MOTOR2_No017.PCONF.Modeswitches.sw14 := FALSE;
   MOTOR2_No017.PCONF.Modeswitches.sw15 := FALSE;
   MOTOR2_No017.PCONF.DlyTCmd := T#0MS;
   MOTOR2_No017.PCONF.DlyTBlackout := T#0MS;
   MOTOR2_No017.PCONF.DlyTExtFault := T#0MS;
   MOTOR2_No017.PCONF.DlyTFeedback := T#0MS;
   MOTOR2_No017.PCONF.DlyTActFault := T#0MS;
   MOTOR2_No017.PCONF.DlyTAutoAl := T#0MS;
   MOTOR2_No017.PCONF.DlyTRestart := T#0MS;
   MOTOR2_No017.PCONF.DlyTChg12 := T#0MS;
   MOTOR2_No017.PCONF.DlyTChg21 := T#0MS;
   MOTOR2_No018.System := W#16#0;
   MOTOR2_No018.CmdOS := W#16#0;
   MOTOR2_No018.MirrorCmdOS := W#16#0;
   MOTOR2_No018.Test := W#16#0;
   MOTOR2_No018.AlarmOS := W#16#0;
   MOTOR2_No018.StatusOS := W#16#0;
   MOTOR2_No018.SysStatusOS := W#16#0;
   MOTOR2_No018.Status1 := W#16#0;
   MOTOR2_No018.Status2 := W#16#0;
   MOTOR2_No018.Status3 := B#16#0;
   MOTOR2_No018.InputEdges := B#16#0;
   MOTOR2_No018.AutoEdges := W#16#0;
   MOTOR2_No018.DataTimeCmd.StartTime := L#0;
   MOTOR2_No018.DataTimeCmd.StartEdge := FALSE;
   MOTOR2_No018.DataTimeChg12.StartTime := L#0;
   MOTOR2_No018.DataTimeChg12.StartEdge := FALSE;
   MOTOR2_No018.DataTimeChg21.StartTime := L#0;
   MOTOR2_No018.DataTimeChg21.StartEdge := FALSE;
   MOTOR2_No018.DataTimeBlackout.StartTime := L#0;
   MOTOR2_No018.DataTimeBlackout.StartEdge := FALSE;
   MOTOR2_No018.DataTimeActFault.StartTime := L#0;
   MOTOR2_No018.DataTimeActFault.StartEdge := FALSE;
   MOTOR2_No018.DataTimeExtFault.StartTime := L#0;
   MOTOR2_No018.DataTimeExtFault.StartEdge := FALSE;
   MOTOR2_No018.DataTimeFeedback.StartTime := L#0;
   MOTOR2_No018.DataTimeFeedback.StartEdge := FALSE;
   MOTOR2_No018.DataTimeAutoAl.StartTime := L#0;
   MOTOR2_No018.DataTimeAutoAl.StartEdge := FALSE;
   MOTOR2_No018.PCONF.Modeswitches.M0_ConstantOut := FALSE;
   MOTOR2_No018.PCONF.Modeswitches.M1_AutoManLoc := FALSE;
   MOTOR2_No018.PCONF.Modeswitches.M2_NoActFeedFault := FALSE;
   MOTOR2_No018.PCONF.Modeswitches.M3_NoStopIfFault := FALSE;
   MOTOR2_No018.PCONF.Modeswitches.M4_RestrtAftBlack := FALSE;
   MOTOR2_No018.PCONF.Modeswitches.M5_ResetOSonly := FALSE;
   MOTOR2_No018.PCONF.Modeswitches.M6_CmdTimeDly := FALSE;
   MOTOR2_No018.PCONF.Modeswitches.M7_Chg12viaStop := FALSE;
   MOTOR2_No018.PCONF.Modeswitches.M8_Chg21viaStop := FALSE;
   MOTOR2_No018.PCONF.Modeswitches.M9_StopIfAutoFail := FALSE;
   MOTOR2_No018.PCONF.Modeswitches.M10_LockBlockCmd := FALSE;
   MOTOR2_No018.PCONF.Modeswitches.sw11 := FALSE;
   MOTOR2_No018.PCONF.Modeswitches.sw12 := FALSE;
   MOTOR2_No018.PCONF.Modeswitches.sw13 := FALSE;
   MOTOR2_No018.PCONF.Modeswitches.sw14 := FALSE;
   MOTOR2_No018.PCONF.Modeswitches.sw15 := FALSE;
   MOTOR2_No018.PCONF.DlyTCmd := T#0MS;
   MOTOR2_No018.PCONF.DlyTBlackout := T#0MS;
   MOTOR2_No018.PCONF.DlyTExtFault := T#0MS;
   MOTOR2_No018.PCONF.DlyTFeedback := T#0MS;
   MOTOR2_No018.PCONF.DlyTActFault := T#0MS;
   MOTOR2_No018.PCONF.DlyTAutoAl := T#0MS;
   MOTOR2_No018.PCONF.DlyTRestart := T#0MS;
   MOTOR2_No018.PCONF.DlyTChg12 := T#0MS;
   MOTOR2_No018.PCONF.DlyTChg21 := T#0MS;
   MOTOR2_No019.System := W#16#0;
   MOTOR2_No019.CmdOS := W#16#0;
   MOTOR2_No019.MirrorCmdOS := W#16#0;
   MOTOR2_No019.Test := W#16#0;
   MOTOR2_No019.AlarmOS := W#16#0;
   MOTOR2_No019.StatusOS := W#16#0;
   MOTOR2_No019.SysStatusOS := W#16#0;
   MOTOR2_No019.Status1 := W#16#0;
   MOTOR2_No019.Status2 := W#16#0;
   MOTOR2_No019.Status3 := B#16#0;
   MOTOR2_No019.InputEdges := B#16#0;
   MOTOR2_No019.AutoEdges := W#16#0;
   MOTOR2_No019.DataTimeCmd.StartTime := L#0;
   MOTOR2_No019.DataTimeCmd.StartEdge := FALSE;
   MOTOR2_No019.DataTimeChg12.StartTime := L#0;
   MOTOR2_No019.DataTimeChg12.StartEdge := FALSE;
   MOTOR2_No019.DataTimeChg21.StartTime := L#0;
   MOTOR2_No019.DataTimeChg21.StartEdge := FALSE;
   MOTOR2_No019.DataTimeBlackout.StartTime := L#0;
   MOTOR2_No019.DataTimeBlackout.StartEdge := FALSE;
   MOTOR2_No019.DataTimeActFault.StartTime := L#0;
   MOTOR2_No019.DataTimeActFault.StartEdge := FALSE;
   MOTOR2_No019.DataTimeExtFault.StartTime := L#0;
   MOTOR2_No019.DataTimeExtFault.StartEdge := FALSE;
   MOTOR2_No019.DataTimeFeedback.StartTime := L#0;
   MOTOR2_No019.DataTimeFeedback.StartEdge := FALSE;
   MOTOR2_No019.DataTimeAutoAl.StartTime := L#0;
   MOTOR2_No019.DataTimeAutoAl.StartEdge := FALSE;
   MOTOR2_No019.PCONF.Modeswitches.M0_ConstantOut := FALSE;
   MOTOR2_No019.PCONF.Modeswitches.M1_AutoManLoc := FALSE;
   MOTOR2_No019.PCONF.Modeswitches.M2_NoActFeedFault := FALSE;
   MOTOR2_No019.PCONF.Modeswitches.M3_NoStopIfFault := FALSE;
   MOTOR2_No019.PCONF.Modeswitches.M4_RestrtAftBlack := FALSE;
   MOTOR2_No019.PCONF.Modeswitches.M5_ResetOSonly := FALSE;
   MOTOR2_No019.PCONF.Modeswitches.M6_CmdTimeDly := FALSE;
   MOTOR2_No019.PCONF.Modeswitches.M7_Chg12viaStop := FALSE;
   MOTOR2_No019.PCONF.Modeswitches.M8_Chg21viaStop := FALSE;
   MOTOR2_No019.PCONF.Modeswitches.M9_StopIfAutoFail := FALSE;
   MOTOR2_No019.PCONF.Modeswitches.M10_LockBlockCmd := FALSE;
   MOTOR2_No019.PCONF.Modeswitches.sw11 := FALSE;
   MOTOR2_No019.PCONF.Modeswitches.sw12 := FALSE;
   MOTOR2_No019.PCONF.Modeswitches.sw13 := FALSE;
   MOTOR2_No019.PCONF.Modeswitches.sw14 := FALSE;
   MOTOR2_No019.PCONF.Modeswitches.sw15 := FALSE;
   MOTOR2_No019.PCONF.DlyTCmd := T#0MS;
   MOTOR2_No019.PCONF.DlyTBlackout := T#0MS;
   MOTOR2_No019.PCONF.DlyTExtFault := T#0MS;
   MOTOR2_No019.PCONF.DlyTFeedback := T#0MS;
   MOTOR2_No019.PCONF.DlyTActFault := T#0MS;
   MOTOR2_No019.PCONF.DlyTAutoAl := T#0MS;
   MOTOR2_No019.PCONF.DlyTRestart := T#0MS;
   MOTOR2_No019.PCONF.DlyTChg12 := T#0MS;
   MOTOR2_No019.PCONF.DlyTChg21 := T#0MS;
   MOTOR2_No020.System := W#16#0;
   MOTOR2_No020.CmdOS := W#16#0;
   MOTOR2_No020.MirrorCmdOS := W#16#0;
   MOTOR2_No020.Test := W#16#0;
   MOTOR2_No020.AlarmOS := W#16#0;
   MOTOR2_No020.StatusOS := W#16#0;
   MOTOR2_No020.SysStatusOS := W#16#0;
   MOTOR2_No020.Status1 := W#16#0;
   MOTOR2_No020.Status2 := W#16#0;
   MOTOR2_No020.Status3 := B#16#0;
   MOTOR2_No020.InputEdges := B#16#0;
   MOTOR2_No020.AutoEdges := W#16#0;
   MOTOR2_No020.DataTimeCmd.StartTime := L#0;
   MOTOR2_No020.DataTimeCmd.StartEdge := FALSE;
   MOTOR2_No020.DataTimeChg12.StartTime := L#0;
   MOTOR2_No020.DataTimeChg12.StartEdge := FALSE;
   MOTOR2_No020.DataTimeChg21.StartTime := L#0;
   MOTOR2_No020.DataTimeChg21.StartEdge := FALSE;
   MOTOR2_No020.DataTimeBlackout.StartTime := L#0;
   MOTOR2_No020.DataTimeBlackout.StartEdge := FALSE;
   MOTOR2_No020.DataTimeActFault.StartTime := L#0;
   MOTOR2_No020.DataTimeActFault.StartEdge := FALSE;
   MOTOR2_No020.DataTimeExtFault.StartTime := L#0;
   MOTOR2_No020.DataTimeExtFault.StartEdge := FALSE;
   MOTOR2_No020.DataTimeFeedback.StartTime := L#0;
   MOTOR2_No020.DataTimeFeedback.StartEdge := FALSE;
   MOTOR2_No020.DataTimeAutoAl.StartTime := L#0;
   MOTOR2_No020.DataTimeAutoAl.StartEdge := FALSE;
   MOTOR2_No020.PCONF.Modeswitches.M0_ConstantOut := FALSE;
   MOTOR2_No020.PCONF.Modeswitches.M1_AutoManLoc := FALSE;
   MOTOR2_No020.PCONF.Modeswitches.M2_NoActFeedFault := FALSE;
   MOTOR2_No020.PCONF.Modeswitches.M3_NoStopIfFault := FALSE;
   MOTOR2_No020.PCONF.Modeswitches.M4_RestrtAftBlack := FALSE;
   MOTOR2_No020.PCONF.Modeswitches.M5_ResetOSonly := FALSE;
   MOTOR2_No020.PCONF.Modeswitches.M6_CmdTimeDly := FALSE;
   MOTOR2_No020.PCONF.Modeswitches.M7_Chg12viaStop := FALSE;
   MOTOR2_No020.PCONF.Modeswitches.M8_Chg21viaStop := FALSE;
   MOTOR2_No020.PCONF.Modeswitches.M9_StopIfAutoFail := FALSE;
   MOTOR2_No020.PCONF.Modeswitches.M10_LockBlockCmd := FALSE;
   MOTOR2_No020.PCONF.Modeswitches.sw11 := FALSE;
   MOTOR2_No020.PCONF.Modeswitches.sw12 := FALSE;
   MOTOR2_No020.PCONF.Modeswitches.sw13 := FALSE;
   MOTOR2_No020.PCONF.Modeswitches.sw14 := FALSE;
   MOTOR2_No020.PCONF.Modeswitches.sw15 := FALSE;
   MOTOR2_No020.PCONF.DlyTCmd := T#0MS;
   MOTOR2_No020.PCONF.DlyTBlackout := T#0MS;
   MOTOR2_No020.PCONF.DlyTExtFault := T#0MS;
   MOTOR2_No020.PCONF.DlyTFeedback := T#0MS;
   MOTOR2_No020.PCONF.DlyTActFault := T#0MS;
   MOTOR2_No020.PCONF.DlyTAutoAl := T#0MS;
   MOTOR2_No020.PCONF.DlyTRestart := T#0MS;
   MOTOR2_No020.PCONF.DlyTChg12 := T#0MS;
   MOTOR2_No020.PCONF.DlyTChg21 := T#0MS;
   MOTOR2_No021.System := W#16#0;
   MOTOR2_No021.CmdOS := W#16#0;
   MOTOR2_No021.MirrorCmdOS := W#16#0;
   MOTOR2_No021.Test := W#16#0;
   MOTOR2_No021.AlarmOS := W#16#0;
   MOTOR2_No021.StatusOS := W#16#0;
   MOTOR2_No021.SysStatusOS := W#16#0;
   MOTOR2_No021.Status1 := W#16#0;
   MOTOR2_No021.Status2 := W#16#0;
   MOTOR2_No021.Status3 := B#16#0;
   MOTOR2_No021.InputEdges := B#16#0;
   MOTOR2_No021.AutoEdges := W#16#0;
   MOTOR2_No021.DataTimeCmd.StartTime := L#0;
   MOTOR2_No021.DataTimeCmd.StartEdge := FALSE;
   MOTOR2_No021.DataTimeChg12.StartTime := L#0;
   MOTOR2_No021.DataTimeChg12.StartEdge := FALSE;
   MOTOR2_No021.DataTimeChg21.StartTime := L#0;
   MOTOR2_No021.DataTimeChg21.StartEdge := FALSE;
   MOTOR2_No021.DataTimeBlackout.StartTime := L#0;
   MOTOR2_No021.DataTimeBlackout.StartEdge := FALSE;
   MOTOR2_No021.DataTimeActFault.StartTime := L#0;
   MOTOR2_No021.DataTimeActFault.StartEdge := FALSE;
   MOTOR2_No021.DataTimeExtFault.StartTime := L#0;
   MOTOR2_No021.DataTimeExtFault.StartEdge := FALSE;
   MOTOR2_No021.DataTimeFeedback.StartTime := L#0;
   MOTOR2_No021.DataTimeFeedback.StartEdge := FALSE;
   MOTOR2_No021.DataTimeAutoAl.StartTime := L#0;
   MOTOR2_No021.DataTimeAutoAl.StartEdge := FALSE;
   MOTOR2_No021.PCONF.Modeswitches.M0_ConstantOut := FALSE;
   MOTOR2_No021.PCONF.Modeswitches.M1_AutoManLoc := FALSE;
   MOTOR2_No021.PCONF.Modeswitches.M2_NoActFeedFault := FALSE;
   MOTOR2_No021.PCONF.Modeswitches.M3_NoStopIfFault := FALSE;
   MOTOR2_No021.PCONF.Modeswitches.M4_RestrtAftBlack := FALSE;
   MOTOR2_No021.PCONF.Modeswitches.M5_ResetOSonly := FALSE;
   MOTOR2_No021.PCONF.Modeswitches.M6_CmdTimeDly := FALSE;
   MOTOR2_No021.PCONF.Modeswitches.M7_Chg12viaStop := FALSE;
   MOTOR2_No021.PCONF.Modeswitches.M8_Chg21viaStop := FALSE;
   MOTOR2_No021.PCONF.Modeswitches.M9_StopIfAutoFail := FALSE;
   MOTOR2_No021.PCONF.Modeswitches.M10_LockBlockCmd := FALSE;
   MOTOR2_No021.PCONF.Modeswitches.sw11 := FALSE;
   MOTOR2_No021.PCONF.Modeswitches.sw12 := FALSE;
   MOTOR2_No021.PCONF.Modeswitches.sw13 := FALSE;
   MOTOR2_No021.PCONF.Modeswitches.sw14 := FALSE;
   MOTOR2_No021.PCONF.Modeswitches.sw15 := FALSE;
   MOTOR2_No021.PCONF.DlyTCmd := T#0MS;
   MOTOR2_No021.PCONF.DlyTBlackout := T#0MS;
   MOTOR2_No021.PCONF.DlyTExtFault := T#0MS;
   MOTOR2_No021.PCONF.DlyTFeedback := T#0MS;
   MOTOR2_No021.PCONF.DlyTActFault := T#0MS;
   MOTOR2_No021.PCONF.DlyTAutoAl := T#0MS;
   MOTOR2_No021.PCONF.DlyTRestart := T#0MS;
   MOTOR2_No021.PCONF.DlyTChg12 := T#0MS;
   MOTOR2_No021.PCONF.DlyTChg21 := T#0MS;
   MOTOR2_No022.System := W#16#0;
   MOTOR2_No022.CmdOS := W#16#0;
   MOTOR2_No022.MirrorCmdOS := W#16#0;
   MOTOR2_No022.Test := W#16#0;
   MOTOR2_No022.AlarmOS := W#16#0;
   MOTOR2_No022.StatusOS := W#16#0;
   MOTOR2_No022.SysStatusOS := W#16#0;
   MOTOR2_No022.Status1 := W#16#0;
   MOTOR2_No022.Status2 := W#16#0;
   MOTOR2_No022.Status3 := B#16#0;
   MOTOR2_No022.InputEdges := B#16#0;
   MOTOR2_No022.AutoEdges := W#16#0;
   MOTOR2_No022.DataTimeCmd.StartTime := L#0;
   MOTOR2_No022.DataTimeCmd.StartEdge := FALSE;
   MOTOR2_No022.DataTimeChg12.StartTime := L#0;
   MOTOR2_No022.DataTimeChg12.StartEdge := FALSE;
   MOTOR2_No022.DataTimeChg21.StartTime := L#0;
   MOTOR2_No022.DataTimeChg21.StartEdge := FALSE;
   MOTOR2_No022.DataTimeBlackout.StartTime := L#0;
   MOTOR2_No022.DataTimeBlackout.StartEdge := FALSE;
   MOTOR2_No022.DataTimeActFault.StartTime := L#0;
   MOTOR2_No022.DataTimeActFault.StartEdge := FALSE;
   MOTOR2_No022.DataTimeExtFault.StartTime := L#0;
   MOTOR2_No022.DataTimeExtFault.StartEdge := FALSE;
   MOTOR2_No022.DataTimeFeedback.StartTime := L#0;
   MOTOR2_No022.DataTimeFeedback.StartEdge := FALSE;
   MOTOR2_No022.DataTimeAutoAl.StartTime := L#0;
   MOTOR2_No022.DataTimeAutoAl.StartEdge := FALSE;
   MOTOR2_No022.PCONF.Modeswitches.M0_ConstantOut := FALSE;
   MOTOR2_No022.PCONF.Modeswitches.M1_AutoManLoc := FALSE;
   MOTOR2_No022.PCONF.Modeswitches.M2_NoActFeedFault := FALSE;
   MOTOR2_No022.PCONF.Modeswitches.M3_NoStopIfFault := FALSE;
   MOTOR2_No022.PCONF.Modeswitches.M4_RestrtAftBlack := FALSE;
   MOTOR2_No022.PCONF.Modeswitches.M5_ResetOSonly := FALSE;
   MOTOR2_No022.PCONF.Modeswitches.M6_CmdTimeDly := FALSE;
   MOTOR2_No022.PCONF.Modeswitches.M7_Chg12viaStop := FALSE;
   MOTOR2_No022.PCONF.Modeswitches.M8_Chg21viaStop := FALSE;
   MOTOR2_No022.PCONF.Modeswitches.M9_StopIfAutoFail := FALSE;
   MOTOR2_No022.PCONF.Modeswitches.M10_LockBlockCmd := FALSE;
   MOTOR2_No022.PCONF.Modeswitches.sw11 := FALSE;
   MOTOR2_No022.PCONF.Modeswitches.sw12 := FALSE;
   MOTOR2_No022.PCONF.Modeswitches.sw13 := FALSE;
   MOTOR2_No022.PCONF.Modeswitches.sw14 := FALSE;
   MOTOR2_No022.PCONF.Modeswitches.sw15 := FALSE;
   MOTOR2_No022.PCONF.DlyTCmd := T#0MS;
   MOTOR2_No022.PCONF.DlyTBlackout := T#0MS;
   MOTOR2_No022.PCONF.DlyTExtFault := T#0MS;
   MOTOR2_No022.PCONF.DlyTFeedback := T#0MS;
   MOTOR2_No022.PCONF.DlyTActFault := T#0MS;
   MOTOR2_No022.PCONF.DlyTAutoAl := T#0MS;
   MOTOR2_No022.PCONF.DlyTRestart := T#0MS;
   MOTOR2_No022.PCONF.DlyTChg12 := T#0MS;
   MOTOR2_No022.PCONF.DlyTChg21 := T#0MS;
   MOTOR2_No023.System := W#16#0;
   MOTOR2_No023.CmdOS := W#16#0;
   MOTOR2_No023.MirrorCmdOS := W#16#0;
   MOTOR2_No023.Test := W#16#0;
   MOTOR2_No023.AlarmOS := W#16#0;
   MOTOR2_No023.StatusOS := W#16#0;
   MOTOR2_No023.SysStatusOS := W#16#0;
   MOTOR2_No023.Status1 := W#16#0;
   MOTOR2_No023.Status2 := W#16#0;
   MOTOR2_No023.Status3 := B#16#0;
   MOTOR2_No023.InputEdges := B#16#0;
   MOTOR2_No023.AutoEdges := W#16#0;
   MOTOR2_No023.DataTimeCmd.StartTime := L#0;
   MOTOR2_No023.DataTimeCmd.StartEdge := FALSE;
   MOTOR2_No023.DataTimeChg12.StartTime := L#0;
   MOTOR2_No023.DataTimeChg12.StartEdge := FALSE;
   MOTOR2_No023.DataTimeChg21.StartTime := L#0;
   MOTOR2_No023.DataTimeChg21.StartEdge := FALSE;
   MOTOR2_No023.DataTimeBlackout.StartTime := L#0;
   MOTOR2_No023.DataTimeBlackout.StartEdge := FALSE;
   MOTOR2_No023.DataTimeActFault.StartTime := L#0;
   MOTOR2_No023.DataTimeActFault.StartEdge := FALSE;
   MOTOR2_No023.DataTimeExtFault.StartTime := L#0;
   MOTOR2_No023.DataTimeExtFault.StartEdge := FALSE;
   MOTOR2_No023.DataTimeFeedback.StartTime := L#0;
   MOTOR2_No023.DataTimeFeedback.StartEdge := FALSE;
   MOTOR2_No023.DataTimeAutoAl.StartTime := L#0;
   MOTOR2_No023.DataTimeAutoAl.StartEdge := FALSE;
   MOTOR2_No023.PCONF.Modeswitches.M0_ConstantOut := FALSE;
   MOTOR2_No023.PCONF.Modeswitches.M1_AutoManLoc := FALSE;
   MOTOR2_No023.PCONF.Modeswitches.M2_NoActFeedFault := FALSE;
   MOTOR2_No023.PCONF.Modeswitches.M3_NoStopIfFault := FALSE;
   MOTOR2_No023.PCONF.Modeswitches.M4_RestrtAftBlack := FALSE;
   MOTOR2_No023.PCONF.Modeswitches.M5_ResetOSonly := FALSE;
   MOTOR2_No023.PCONF.Modeswitches.M6_CmdTimeDly := FALSE;
   MOTOR2_No023.PCONF.Modeswitches.M7_Chg12viaStop := FALSE;
   MOTOR2_No023.PCONF.Modeswitches.M8_Chg21viaStop := FALSE;
   MOTOR2_No023.PCONF.Modeswitches.M9_StopIfAutoFail := FALSE;
   MOTOR2_No023.PCONF.Modeswitches.M10_LockBlockCmd := FALSE;
   MOTOR2_No023.PCONF.Modeswitches.sw11 := FALSE;
   MOTOR2_No023.PCONF.Modeswitches.sw12 := FALSE;
   MOTOR2_No023.PCONF.Modeswitches.sw13 := FALSE;
   MOTOR2_No023.PCONF.Modeswitches.sw14 := FALSE;
   MOTOR2_No023.PCONF.Modeswitches.sw15 := FALSE;
   MOTOR2_No023.PCONF.DlyTCmd := T#0MS;
   MOTOR2_No023.PCONF.DlyTBlackout := T#0MS;
   MOTOR2_No023.PCONF.DlyTExtFault := T#0MS;
   MOTOR2_No023.PCONF.DlyTFeedback := T#0MS;
   MOTOR2_No023.PCONF.DlyTActFault := T#0MS;
   MOTOR2_No023.PCONF.DlyTAutoAl := T#0MS;
   MOTOR2_No023.PCONF.DlyTRestart := T#0MS;
   MOTOR2_No023.PCONF.DlyTChg12 := T#0MS;
   MOTOR2_No023.PCONF.DlyTChg21 := T#0MS;
   MOTOR2_No024.System := W#16#0;
   MOTOR2_No024.CmdOS := W#16#0;
   MOTOR2_No024.MirrorCmdOS := W#16#0;
   MOTOR2_No024.Test := W#16#0;
   MOTOR2_No024.AlarmOS := W#16#0;
   MOTOR2_No024.StatusOS := W#16#0;
   MOTOR2_No024.SysStatusOS := W#16#0;
   MOTOR2_No024.Status1 := W#16#0;
   MOTOR2_No024.Status2 := W#16#0;
   MOTOR2_No024.Status3 := B#16#0;
   MOTOR2_No024.InputEdges := B#16#0;
   MOTOR2_No024.AutoEdges := W#16#0;
   MOTOR2_No024.DataTimeCmd.StartTime := L#0;
   MOTOR2_No024.DataTimeCmd.StartEdge := FALSE;
   MOTOR2_No024.DataTimeChg12.StartTime := L#0;
   MOTOR2_No024.DataTimeChg12.StartEdge := FALSE;
   MOTOR2_No024.DataTimeChg21.StartTime := L#0;
   MOTOR2_No024.DataTimeChg21.StartEdge := FALSE;
   MOTOR2_No024.DataTimeBlackout.StartTime := L#0;
   MOTOR2_No024.DataTimeBlackout.StartEdge := FALSE;
   MOTOR2_No024.DataTimeActFault.StartTime := L#0;
   MOTOR2_No024.DataTimeActFault.StartEdge := FALSE;
   MOTOR2_No024.DataTimeExtFault.StartTime := L#0;
   MOTOR2_No024.DataTimeExtFault.StartEdge := FALSE;
   MOTOR2_No024.DataTimeFeedback.StartTime := L#0;
   MOTOR2_No024.DataTimeFeedback.StartEdge := FALSE;
   MOTOR2_No024.DataTimeAutoAl.StartTime := L#0;
   MOTOR2_No024.DataTimeAutoAl.StartEdge := FALSE;
   MOTOR2_No024.PCONF.Modeswitches.M0_ConstantOut := FALSE;
   MOTOR2_No024.PCONF.Modeswitches.M1_AutoManLoc := FALSE;
   MOTOR2_No024.PCONF.Modeswitches.M2_NoActFeedFault := FALSE;
   MOTOR2_No024.PCONF.Modeswitches.M3_NoStopIfFault := FALSE;
   MOTOR2_No024.PCONF.Modeswitches.M4_RestrtAftBlack := FALSE;
   MOTOR2_No024.PCONF.Modeswitches.M5_ResetOSonly := FALSE;
   MOTOR2_No024.PCONF.Modeswitches.M6_CmdTimeDly := FALSE;
   MOTOR2_No024.PCONF.Modeswitches.M7_Chg12viaStop := FALSE;
   MOTOR2_No024.PCONF.Modeswitches.M8_Chg21viaStop := FALSE;
   MOTOR2_No024.PCONF.Modeswitches.M9_StopIfAutoFail := FALSE;
   MOTOR2_No024.PCONF.Modeswitches.M10_LockBlockCmd := FALSE;
   MOTOR2_No024.PCONF.Modeswitches.sw11 := FALSE;
   MOTOR2_No024.PCONF.Modeswitches.sw12 := FALSE;
   MOTOR2_No024.PCONF.Modeswitches.sw13 := FALSE;
   MOTOR2_No024.PCONF.Modeswitches.sw14 := FALSE;
   MOTOR2_No024.PCONF.Modeswitches.sw15 := FALSE;
   MOTOR2_No024.PCONF.DlyTCmd := T#0MS;
   MOTOR2_No024.PCONF.DlyTBlackout := T#0MS;
   MOTOR2_No024.PCONF.DlyTExtFault := T#0MS;
   MOTOR2_No024.PCONF.DlyTFeedback := T#0MS;
   MOTOR2_No024.PCONF.DlyTActFault := T#0MS;
   MOTOR2_No024.PCONF.DlyTAutoAl := T#0MS;
   MOTOR2_No024.PCONF.DlyTRestart := T#0MS;
   MOTOR2_No024.PCONF.DlyTChg12 := T#0MS;
   MOTOR2_No024.PCONF.DlyTChg21 := T#0MS;
   MOTOR2_No025.System := W#16#0;
   MOTOR2_No025.CmdOS := W#16#0;
   MOTOR2_No025.MirrorCmdOS := W#16#0;
   MOTOR2_No025.Test := W#16#0;
   MOTOR2_No025.AlarmOS := W#16#0;
   MOTOR2_No025.StatusOS := W#16#0;
   MOTOR2_No025.SysStatusOS := W#16#0;
   MOTOR2_No025.Status1 := W#16#0;
   MOTOR2_No025.Status2 := W#16#0;
   MOTOR2_No025.Status3 := B#16#0;
   MOTOR2_No025.InputEdges := B#16#0;
   MOTOR2_No025.AutoEdges := W#16#0;
   MOTOR2_No025.DataTimeCmd.StartTime := L#0;
   MOTOR2_No025.DataTimeCmd.StartEdge := FALSE;
   MOTOR2_No025.DataTimeChg12.StartTime := L#0;
   MOTOR2_No025.DataTimeChg12.StartEdge := FALSE;
   MOTOR2_No025.DataTimeChg21.StartTime := L#0;
   MOTOR2_No025.DataTimeChg21.StartEdge := FALSE;
   MOTOR2_No025.DataTimeBlackout.StartTime := L#0;
   MOTOR2_No025.DataTimeBlackout.StartEdge := FALSE;
   MOTOR2_No025.DataTimeActFault.StartTime := L#0;
   MOTOR2_No025.DataTimeActFault.StartEdge := FALSE;
   MOTOR2_No025.DataTimeExtFault.StartTime := L#0;
   MOTOR2_No025.DataTimeExtFault.StartEdge := FALSE;
   MOTOR2_No025.DataTimeFeedback.StartTime := L#0;
   MOTOR2_No025.DataTimeFeedback.StartEdge := FALSE;
   MOTOR2_No025.DataTimeAutoAl.StartTime := L#0;
   MOTOR2_No025.DataTimeAutoAl.StartEdge := FALSE;
   MOTOR2_No025.PCONF.Modeswitches.M0_ConstantOut := FALSE;
   MOTOR2_No025.PCONF.Modeswitches.M1_AutoManLoc := FALSE;
   MOTOR2_No025.PCONF.Modeswitches.M2_NoActFeedFault := FALSE;
   MOTOR2_No025.PCONF.Modeswitches.M3_NoStopIfFault := FALSE;
   MOTOR2_No025.PCONF.Modeswitches.M4_RestrtAftBlack := FALSE;
   MOTOR2_No025.PCONF.Modeswitches.M5_ResetOSonly := FALSE;
   MOTOR2_No025.PCONF.Modeswitches.M6_CmdTimeDly := FALSE;
   MOTOR2_No025.PCONF.Modeswitches.M7_Chg12viaStop := FALSE;
   MOTOR2_No025.PCONF.Modeswitches.M8_Chg21viaStop := FALSE;
   MOTOR2_No025.PCONF.Modeswitches.M9_StopIfAutoFail := FALSE;
   MOTOR2_No025.PCONF.Modeswitches.M10_LockBlockCmd := FALSE;
   MOTOR2_No025.PCONF.Modeswitches.sw11 := FALSE;
   MOTOR2_No025.PCONF.Modeswitches.sw12 := FALSE;
   MOTOR2_No025.PCONF.Modeswitches.sw13 := FALSE;
   MOTOR2_No025.PCONF.Modeswitches.sw14 := FALSE;
   MOTOR2_No025.PCONF.Modeswitches.sw15 := FALSE;
   MOTOR2_No025.PCONF.DlyTCmd := T#0MS;
   MOTOR2_No025.PCONF.DlyTBlackout := T#0MS;
   MOTOR2_No025.PCONF.DlyTExtFault := T#0MS;
   MOTOR2_No025.PCONF.DlyTFeedback := T#0MS;
   MOTOR2_No025.PCONF.DlyTActFault := T#0MS;
   MOTOR2_No025.PCONF.DlyTAutoAl := T#0MS;
   MOTOR2_No025.PCONF.DlyTRestart := T#0MS;
   MOTOR2_No025.PCONF.DlyTChg12 := T#0MS;
   MOTOR2_No025.PCONF.DlyTChg21 := T#0MS;
END_DATA_BLOCK

